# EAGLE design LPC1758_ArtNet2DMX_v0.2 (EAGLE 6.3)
Assembly variants: OHNE USB, OHNE VCC2

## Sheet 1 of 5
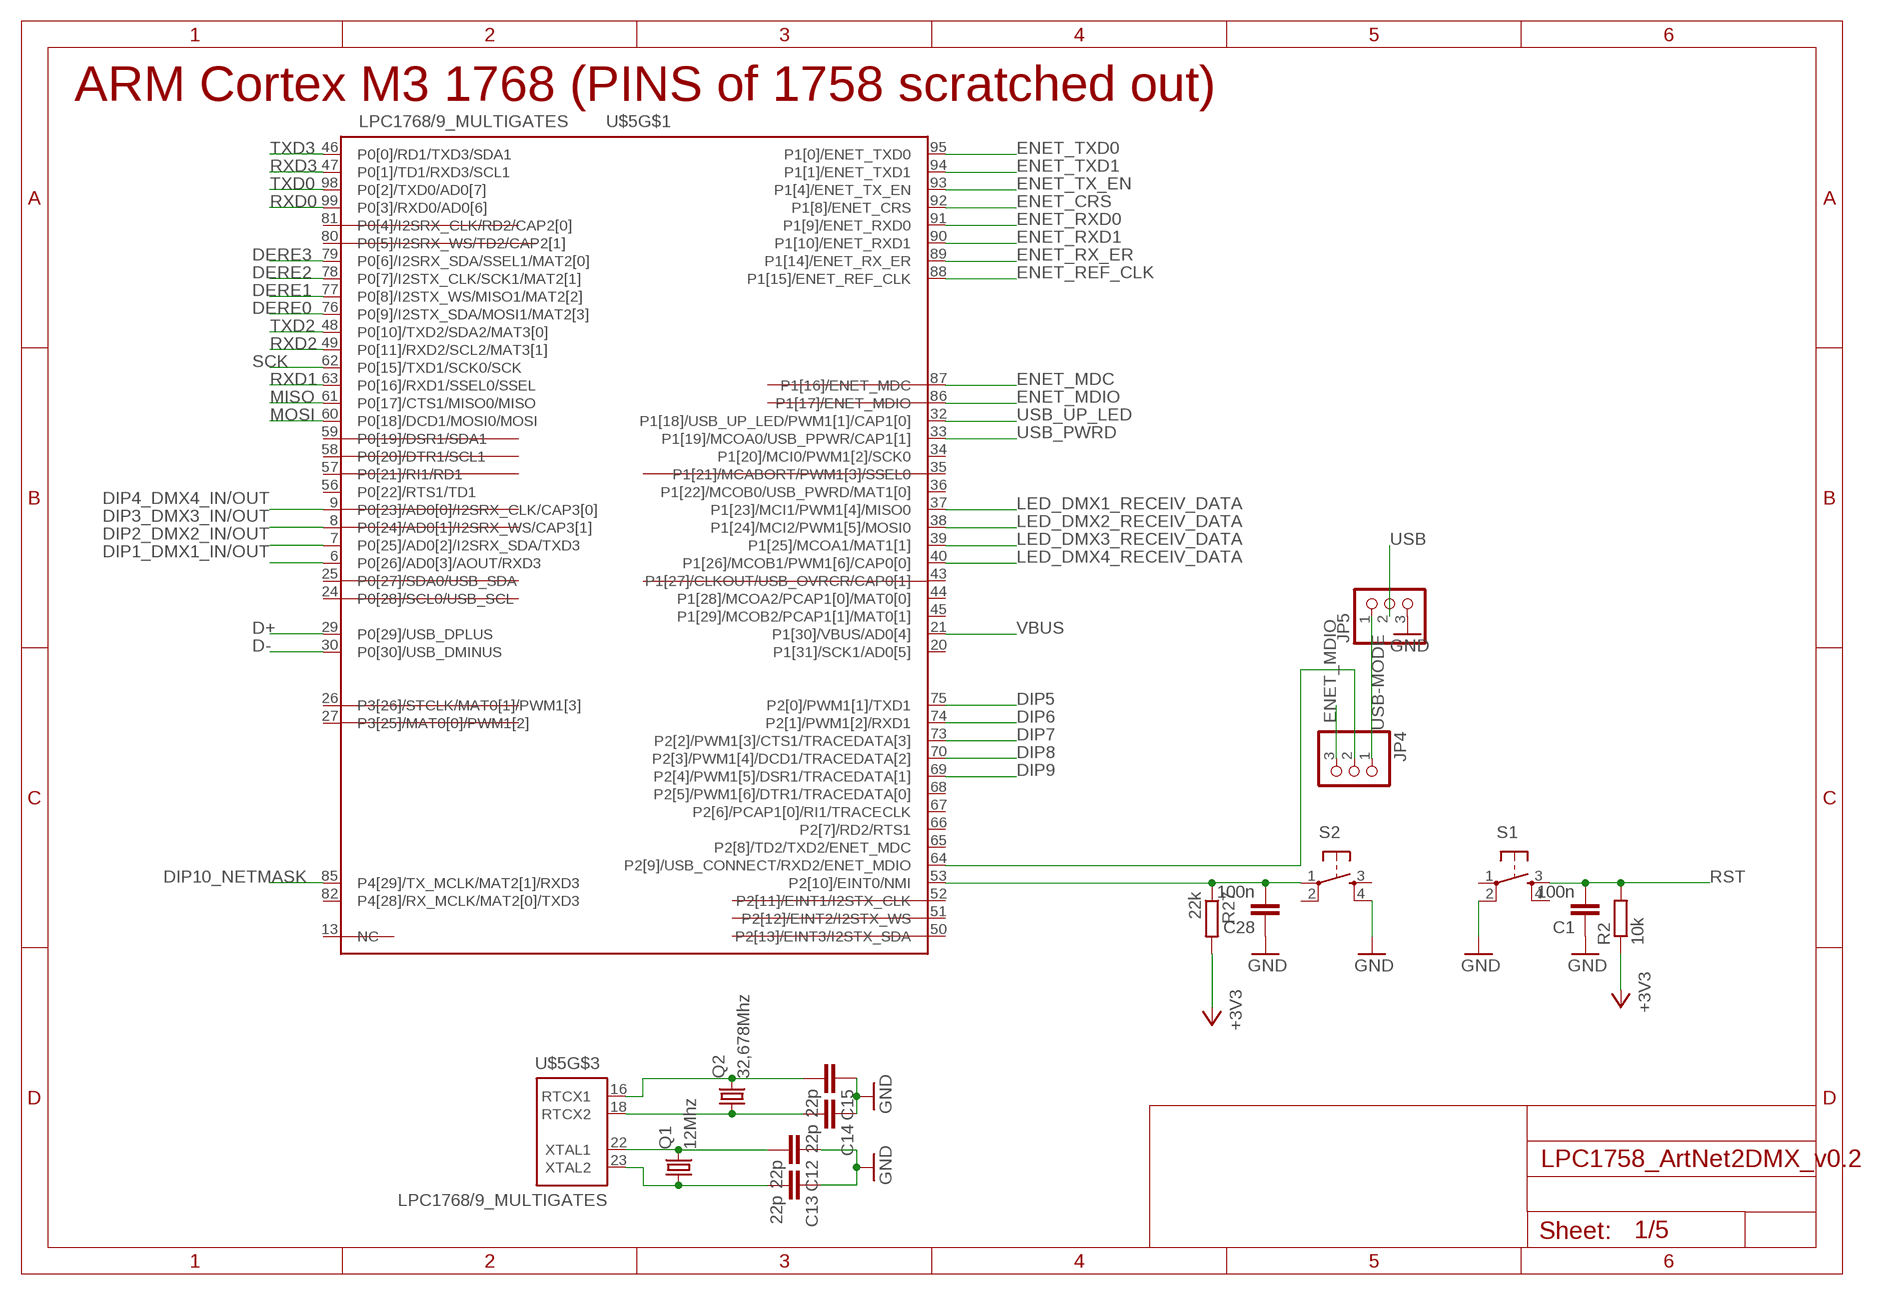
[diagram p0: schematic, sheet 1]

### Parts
C1  100n  C-EUC0805K  [C0805K]
C12  22p  C-EUC0805K  [C0805K]
C13  22p  C-EUC0805K  [C0805K]
C14  22p  C-EUC0805K  [C0805K]
C15  22p  C-EUC0805K  [C0805K]
C28  100n  C-EUC0805K  [C0805K]
JP4  PINHD-1X3_2.54-SMD  [1X03SMD]
JP5  PINHD-1X3_2.54-SMD  [1X03SMD]
Q1  12Mhz  CSM-7X-DU  [CSM-7X-DU]
Q2  32,678Mhz  CSM-7X-DU  [CSM-7X-DU]
R2  10k  R-EU_R0805  [R0805]
R27  22k  R-EU_R0805  [R0805]
S1  TASTER_93XX  [TASTER_93XX]
S2  TASTER_93XX  [TASTER_93XX]
U$5  LPC1768/9_MULTIGATES  [LQFP100-14X14]

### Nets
+3V3: R2.1 R27.2 ; also sheet 2,3,4,5
BUTTON_RESERVE: C28.2 R27.1 S2.1(P) U$5.53(P2[10]/EINT0/NMI)
D+: U$5.29(P0[29]/USB_DPLUS) ; also sheet 4
D-: U$5.30(P0[30]/USB_DMINUS) ; also sheet 4
DERE0: U$5.76(P0[9]/I2STX_SDA/MOSI1/MAT2[3]) ; also sheet 3
DERE1: U$5.77(P0[8]/I2STX_WS/MISO1/MAT2[2]) ; also sheet 3
DERE2: U$5.78(P0[7]/I2STX_CLK/SCK1/MAT2[1]) ; also sheet 3
DERE3: U$5.79(P0[6]/I2SRX_SDA/SSEL1/MAT2[0]) ; also sheet 3
DIP1_DMX1_IN/OUT: U$5.6(P0[26]/AD0[3]/AOUT/RXD3) ; also sheet 3
DIP2_DMX2_IN/OUT: U$5.7(P0[25]/AD0[2]/I2SRX_SDA/TXD3) ; also sheet 3
DIP3_DMX3_IN/OUT: U$5.8(P0[24]/AD0[1]/I2SRX_WS/CAP3[1]) ; also sheet 3
DIP4_DMX4_IN/OUT: U$5.9(P0[23]/AD0[0]/I2SRX_CLK/CAP3[0]) ; also sheet 3
DIP5: U$5.75(P2[0]/PWM1[1]/TXD1) ; also sheet 3
DIP6: U$5.74(P2[1]/PWM1[2]/RXD1) ; also sheet 3
DIP7: U$5.73(P2[2]/PWM1[3]/CTS1/TRACEDATA[3]) ; also sheet 3
DIP8: U$5.70(P2[3]/PWM1[4]/DCD1/TRACEDATA[2]) ; also sheet 3
DIP9: U$5.69(P2[4]/PWM1[5]/DSR1/TRACEDATA[1]) ; also sheet 3
DIP10_NETMASK: U$5.85(P4[29]/TX_MCLK/MAT2[1]/RXD3) ; also sheet 3
ENET_CRS: U$5.92(P1[8]/ENET_CRS) ; also sheet 2
ENET_MDC: U$5.87(P1[16]/ENET_MDC) ; also sheet 2
ENET_MDIO: JP4.3 U$5.86(P1[17]/ENET_MDIO) ; also sheet 2
ENET_MDIO/USB: JP4.2 U$5.64(P2[9]/USB_CONNECT/RXD2/ENET_MDIO)
ENET_REF_CLK: U$5.88(P1[15]/ENET_REF_CLK) ; also sheet 2
ENET_RX_ER: U$5.89(P1[14]/ENET_RX_ER) ; also sheet 2
ENET_RXD0: U$5.91(P1[9]/ENET_RXD0) ; also sheet 2
ENET_RXD1: U$5.90(P1[10]/ENET_RXD1) ; also sheet 2
ENET_TX_EN: U$5.93(P1[4]/ENET_TX_EN) ; also sheet 2
ENET_TXD0: U$5.95(P1[0]/ENET_TXD0) ; also sheet 2
ENET_TXD1: U$5.94(P1[1]/ENET_TXD1) ; also sheet 2
GND: C1.1 C12.1 C13.1 C14.1 C15.1 C28.1 JP5.3 S1.2(P1) S2.4(S1) ; also sheet 2,3,4,5
LED_DMX1_RECEIV_DATA: U$5.37(P1[23]/MCI1/PWM1[4]/MISO0) ; also sheet 3
LED_DMX2_RECEIV_DATA: U$5.38(P1[24]/MCI2/PWM1[5]/MOSI0) ; also sheet 3
LED_DMX3_RECEIV_DATA: U$5.39(P1[25]/MCOA1/MAT1[1]) ; also sheet 3
LED_DMX4_RECEIV_DATA: U$5.40(P1[26]/MCOB1/PWM1[6]/CAP0[0]) ; also sheet 3
MISO: U$5.61(P0[17]/CTS1/MISO0/MISO) ; also sheet 5
MOSI: U$5.60(P0[18]/DCD1/MOSI0/MOSI) ; also sheet 5
N$12: C12.2 Q1.2 U$5.22(XTAL1)
N$13: C13.2 Q1.1 U$5.23(XTAL2)
N$16: C14.2 Q2.1 U$5.18(RTCX2)
N$20: C15.2 Q2.2 U$5.16(RTCX1)
RST: C1.2 R2.2 S1.3(S) ; also sheet 2,5
RXD0: U$5.99(P0[3]/RXD0/AD0[6]) ; also sheet 3
RXD1: U$5.63(P0[16]/RXD1/SSEL0/SSEL) ; also sheet 3
RXD2: U$5.49(P0[11]/RXD2/SCL2/MAT3[1]) ; also sheet 3
RXD3: U$5.47(P0[1]/TD1/RXD3/SCL1) ; also sheet 3
SCK: U$5.62(P0[15]/TXD1/SCK0/SCK) ; also sheet 5
TXD0: U$5.98(P0[2]/TXD0/AD0[7]) ; also sheet 3
TXD2: U$5.48(P0[10]/TXD2/SDA2/MAT3[0]) ; also sheet 3
TXD3: U$5.46(P0[0]/RD1/TXD3/SDA1) ; also sheet 3
USB: JP5.2 ; also sheet 4
USB-MODE: JP4.1 JP5.1
USB_PWRD: U$5.33(P1[19]/MCOA0/USB_PPWR/CAP1[1]) ; also sheet 4
USB_UP_LED: U$5.32(P1[18]/USB_UP_LED/PWM1[1]/CAP1[0]) ; also sheet 4
VBUS: U$5.21(P1[30]/VBUS/AD0[4]) ; also sheet 4
Unconnected: S1.1(P) S1.4(S1) S2.2(P1) S2.3(S) U$5.13(NC) U$5.20(P1[31]/SCK1/AD0[5]) U$5.24(P0[28]/SCL0/USB_SCL) U$5.25(P0[27]/SDA0/USB_SDA) U$5.26(P3[26]/STCLK/MAT0[1]/PWM1[3]) U$5.27(P3[25]/MAT0[0]/PWM1[2]) U$5.34(P1[20]/MCI0/PWM1[2]/SCK0) U$5.35(P1[21]/MCABORT/PWM1[3]/SSEL0) U$5.36(P1[22]/MCOB0/USB_PWRD/MAT1[0]) U$5.43(P1[27]/CLKOUT/USB_OVRCR/CAP0[1]) U$5.44(P1[28]/MCOA2/PCAP1[0]/MAT0[0]) U$5.45(P1[29]/MCOB2/PCAP1[1]/MAT0[1]) U$5.50(P2[13]/EINT3/I2STX_SDA) U$5.51(P2[12]/EINT2/I2STX_WS) U$5.52(P2[11]/EINT1/I2STX_CLK) U$5.56(P0[22]/RTS1/TD1) U$5.57(P0[21]/RI1/RD1) U$5.58(P0[20]/DTR1/SCL1) U$5.59(P0[19]/DSR1/SDA1) U$5.65(P2[8]/TD2/TXD2/ENET_MDC) U$5.66(P2[7]/RD2/RTS1) U$5.67(P2[6]/PCAP1[0]/RI1/TRACECLK) U$5.68(P2[5]/PWM1[6]/DTR1/TRACEDATA[0]) U$5.80(P0[5]/I2SRX_WS/TD2/CAP2[1]) U$5.81(P0[4]/I2SRX_CLK/RD2/CAP2[0]) U$5.82(P4[28]/RX_MCLK/MAT2[0]/TXD3)

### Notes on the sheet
- ARM Cortex M3 1768 (PINS of 1758 scratched out)

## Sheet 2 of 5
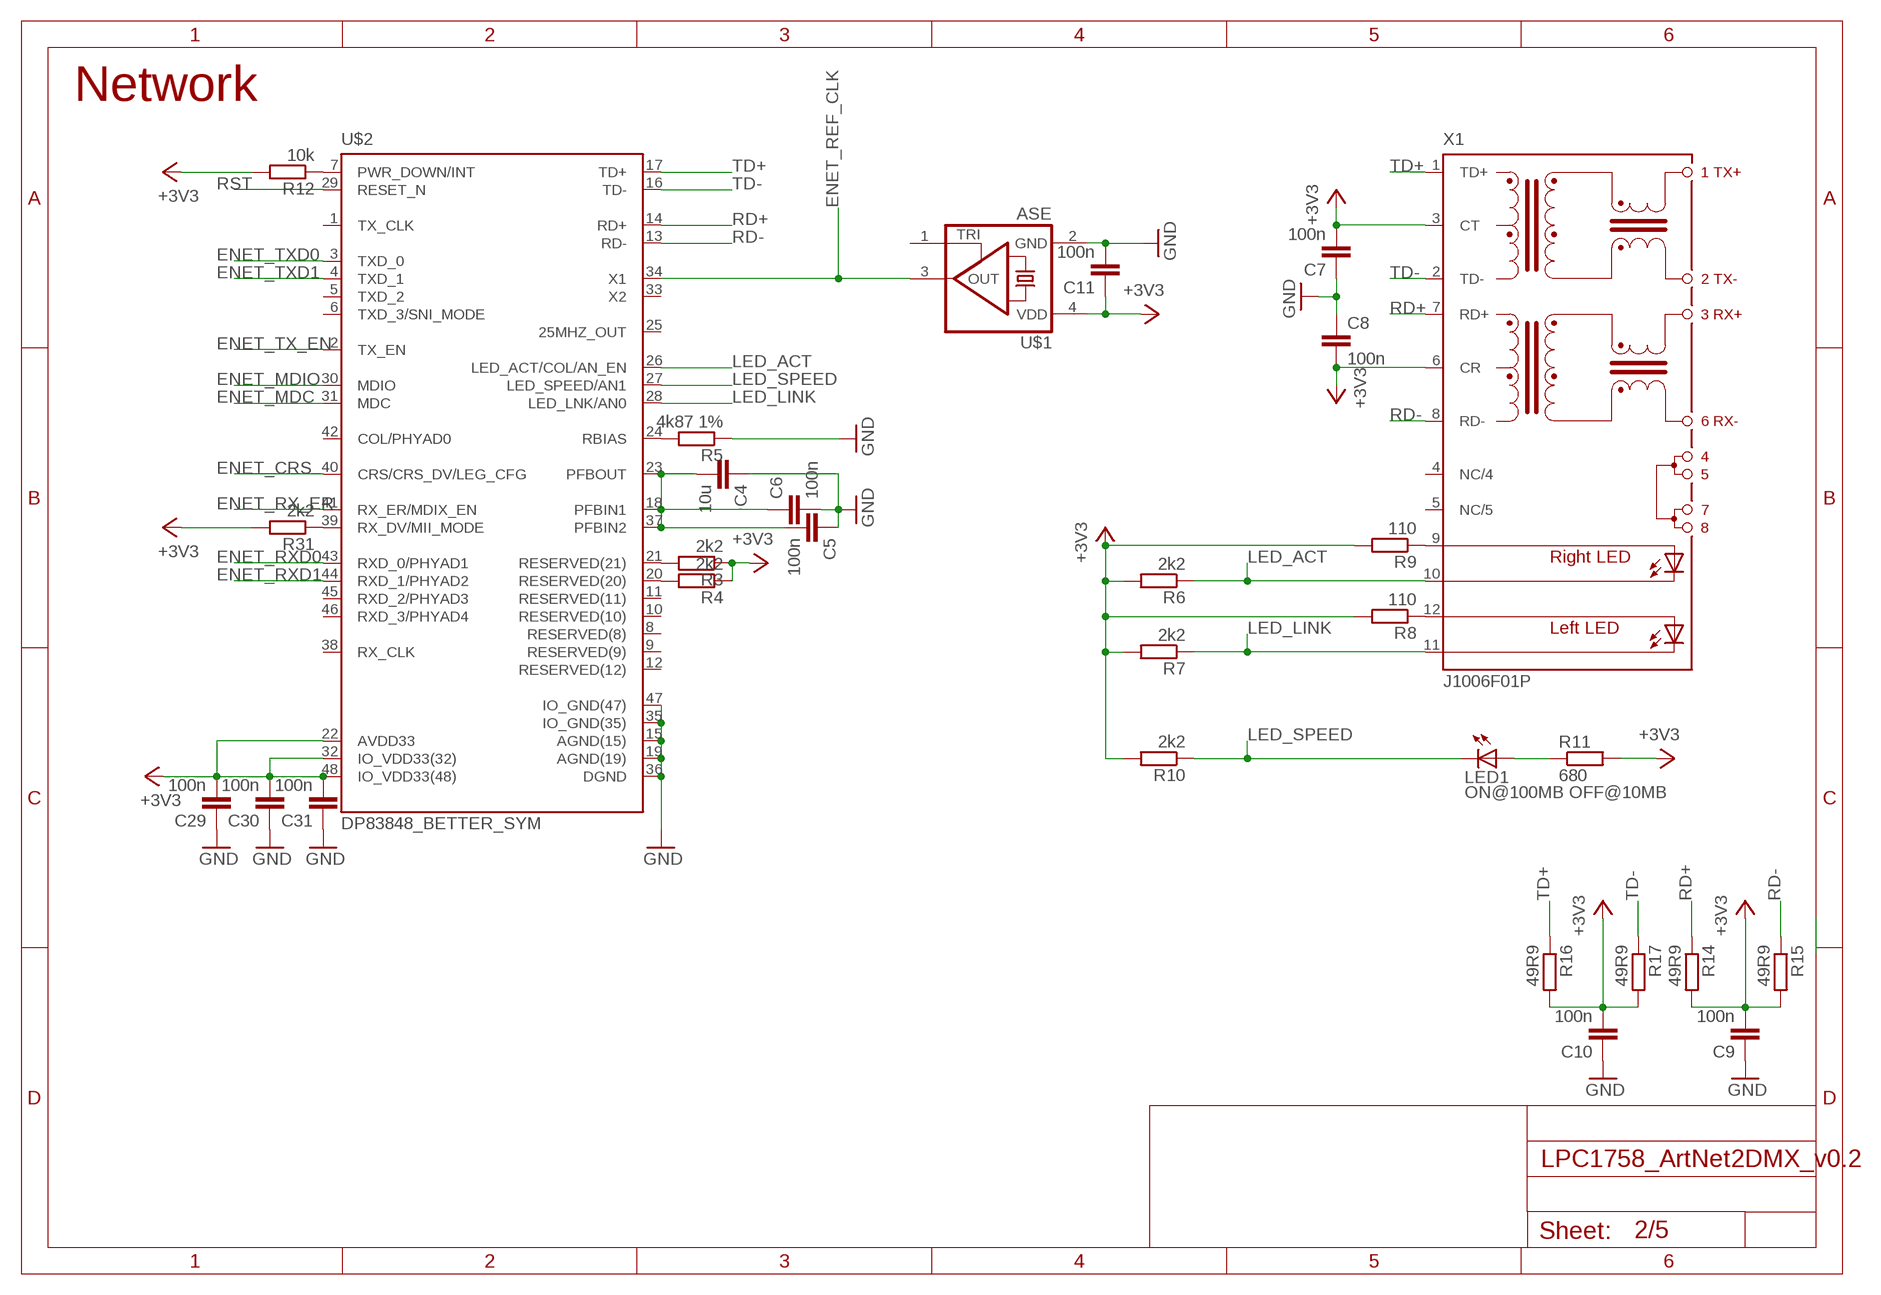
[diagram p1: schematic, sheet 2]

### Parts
C4  10u  C-EUC0805K  [C0805K]
C5  100n  C-EUC0805K  [C0805K]
C6  100n  C-EUC0805K  [C0805K]
C7  100n  C-EUC0805K  [C0805K]
C8  100n  C-EUC0805K  [C0805K]
C9  100n  C-EUC0805K  [C0805K]
C10  100n  C-EUC0805K  [C0805K]
C11  100n  C-EUC0805K  [C0805K]
C29  100n  C-EUC0805K  [C0805K]
C30  100n  C-EUC0805K  [C0805K]
C31  100n  C-EUC0805K  [C0805K]
LED1  ON@100MB OFF@10MB  LEDCHIP-LED0805  [CHIP-LED0805]
R3  2k2  R-EU_R0805  [R0805]
R4  2k2  R-EU_R0805  [R0805]
R5  4k87 1%  R-EU_R0805  [R0805]
R6  2k2  R-EU_R0805  [R0805]
R7  2k2  R-EU_R0805  [R0805]
R8  110  R-EU_R0805  [R0805]
R9  110  R-EU_R0805  [R0805]
R10  2k2  R-EU_R0805  [R0805]
R11  680  R-EU_R0805  [R0805]
R12  10k  R-EU_R0805  [R0805]
R14  49R9  R-EU_R0805  [R0805]
R15  49R9  R-EU_R0805  [R0805]
R16  49R9  R-EU_R0805  [R0805]
R17  49R9  R-EU_R0805  [R0805]
R31  2k2  R-EU_R0805  [R0805]
U$1  ASE  [ASE]
U$2  DP83848_BETTER_SYM  [LQFP48]
X1  J1006F01P  [J1]

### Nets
+3V3: C7.2 C8.2 C9.2 C10.2 C11.1 C29.2 C30.2 C31.2 R3.1 R4.1 R6.2 R7.2 R8.2 R9.2 R10.2 R11.2 R12.2 R14.2 R15.2 R16.2 R17.2 R31.2 U$1.4(VDD) U$2.22(AVDD33) U$2.32(IO_VDD33(32)) U$2.48(IO_VDD33(48)) X1.3(CT) X1.6(CR) ; also sheet 1,3,4,5
ENET_CRS: U$2.40(CRS/CRS_DV/LEG_CFG) ; also sheet 1
ENET_MDC: U$2.31(MDC) ; also sheet 1
ENET_MDIO: U$2.30(MDIO) ; also sheet 1
ENET_REF_CLK: U$1.3(OUT) U$2.34(X1) ; also sheet 1
ENET_RX_ER: U$2.41(RX_ER/MDIX_EN) ; also sheet 1
ENET_RXD0: U$2.43(RXD_0/PHYAD1) ; also sheet 1
ENET_RXD1: U$2.44(RXD_1/PHYAD2) ; also sheet 1
ENET_TX_EN: U$2.2(TX_EN) ; also sheet 1
ENET_TXD0: U$2.3(TXD_0) ; also sheet 1
ENET_TXD1: U$2.4(TXD_1) ; also sheet 1
GND: C4.1 C5.1 C6.2 C7.1 C8.1 C9.1 C10.1 C11.2 C29.1 C30.1 C31.1 R5.1 U$1.2(GND) U$2.15(AGND(15)) U$2.19(AGND(19)) U$2.35(IO_GND(35)) U$2.36(DGND) U$2.47(IO_GND(47)) ; also sheet 1,3,4,5
LED_ACT: R6.1 U$2.26(LED_ACT/COL/AN_EN) X1.10(C-R)
LED_LINK: R7.1 U$2.28(LED_LNK/AN0) X1.11(C-L)
LED_SPEED: LED1.C R10.1 U$2.27(LED_SPEED/AN1)
N$4: R8.1 X1.12(A-L)
N$8: R9.1 X1.9(A-R)
N$9: LED1.A R11.1
N$10: R12.1 U$2.7(PWR_DOWN/INT)
N$14: R3.2 U$2.21(RESERVED(21))
N$15: R4.2 U$2.20(RESERVED(20))
N$17: C4.2 C5.2 C6.1 U$2.18(PFBIN1) U$2.23(PFBOUT) U$2.37(PFBIN2)
N$18: R5.2 U$2.24(RBIAS)
N$19: R31.1 U$2.39(RX_DV/MII_MODE)
RD+: R14.1 U$2.14(RD+) X1.7(RD+)
RD-: R15.1 U$2.13(RD-) X1.8(RD-)
RST: U$2.29(RESET_N) ; also sheet 1,5
TD+: R16.1 U$2.17(TD+) X1.1(TD+)
TD-: R17.1 U$2.16(TD-) X1.2(TD-)
Unconnected: U$1.1(TRI) U$2.1(TX_CLK) U$2.5(TXD_2) U$2.6(TXD_3/SNI_MODE) U$2.8(RESERVED(8)) U$2.9(RESERVED(9)) U$2.10(RESERVED(10)) U$2.11(RESERVED(11)) U$2.12(RESERVED(12)) U$2.25(25MHZ_OUT) U$2.33(X2) U$2.38(RX_CLK) U$2.42(COL/PHYAD0) U$2.45(RXD_2/PHYAD3) U$2.46(RXD_3/PHYAD4) X1.4(NC/4) X1.5(NC/5)

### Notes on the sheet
- Network

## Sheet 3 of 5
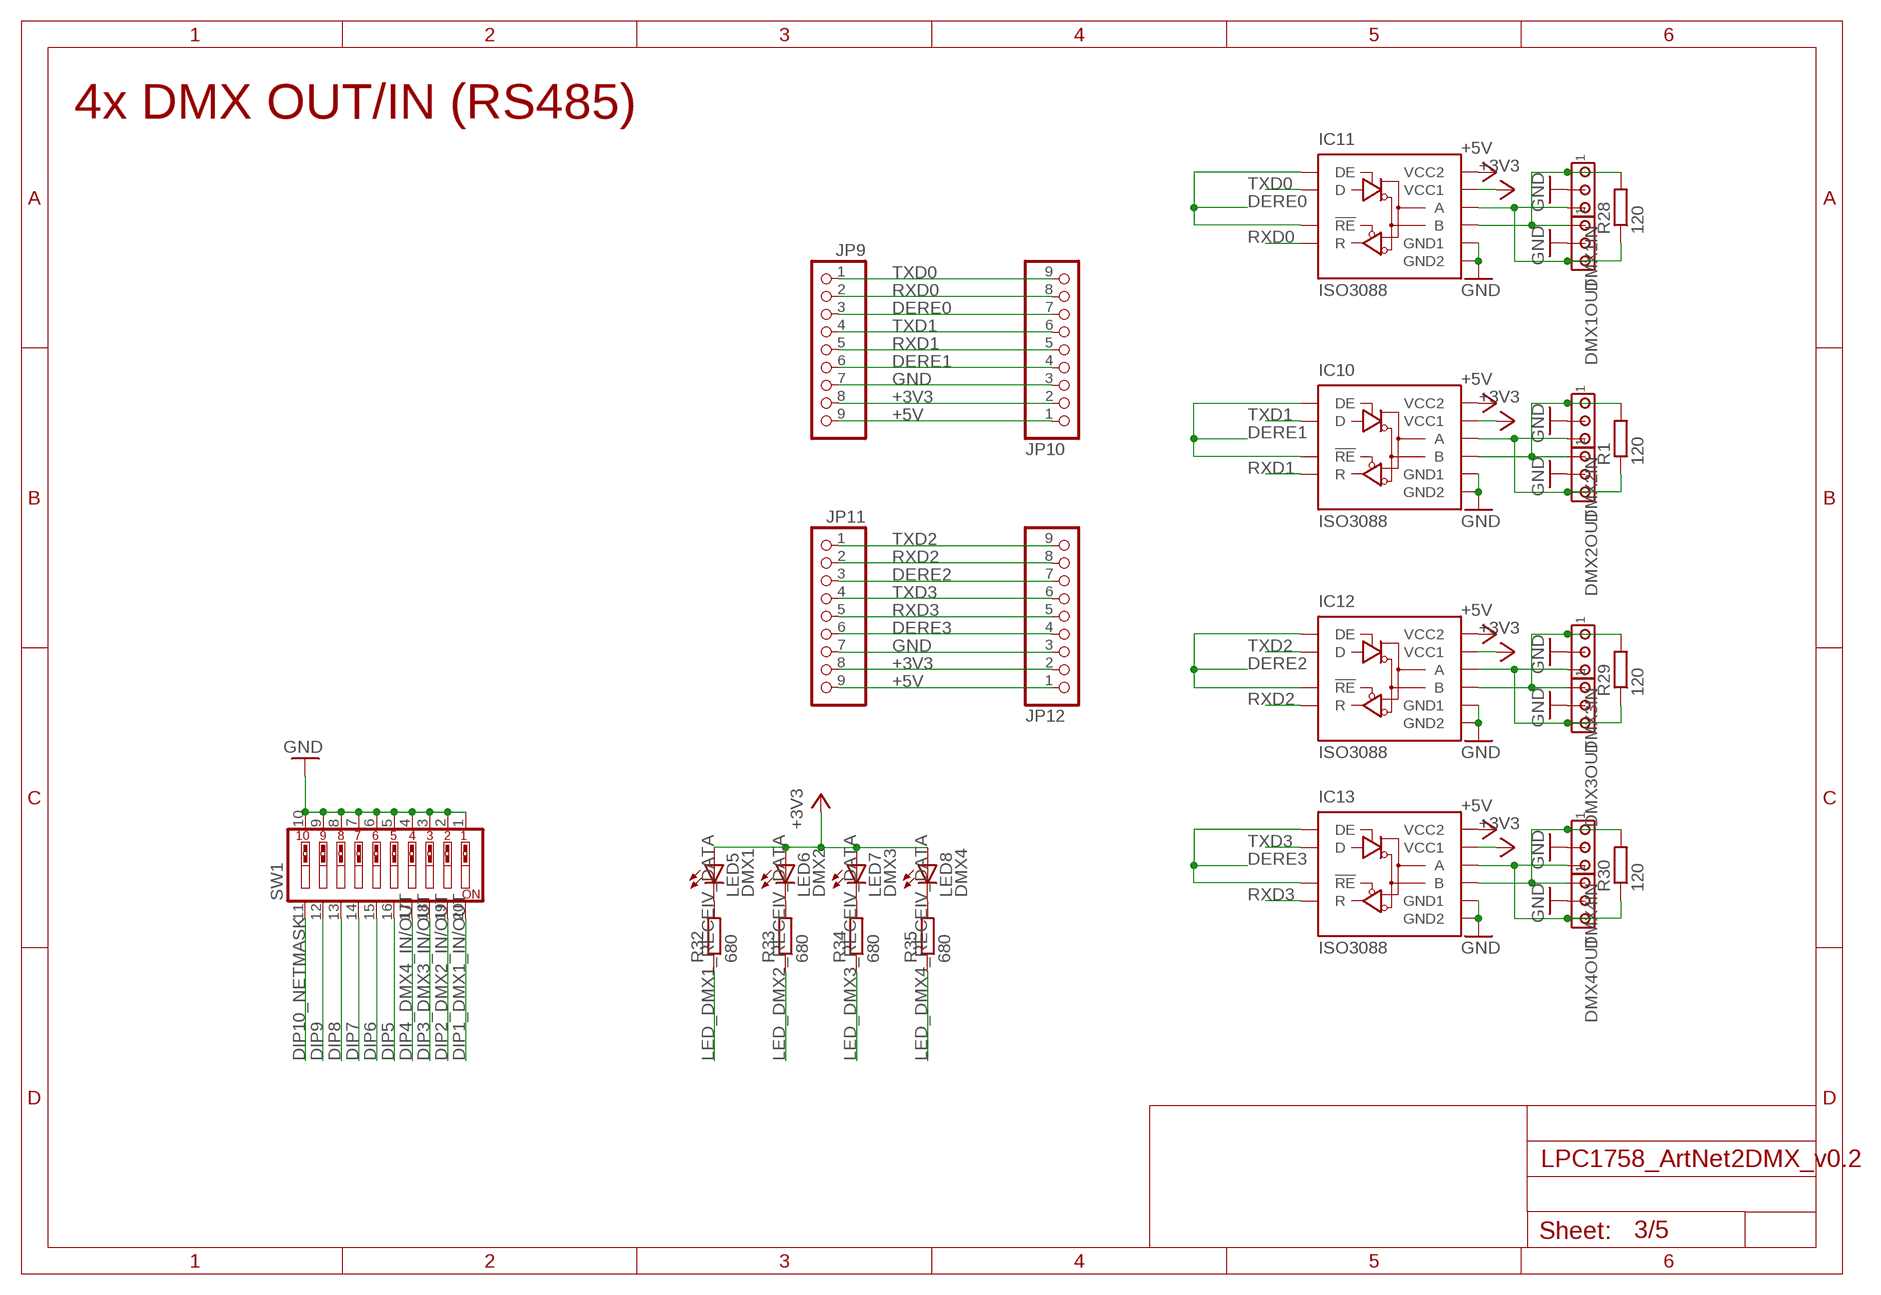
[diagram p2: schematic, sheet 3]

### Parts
DMX1IN  MTA03-100  [10X03MTA]
DMX1OUT  MTA03-100  [10X03MTA]
DMX2IN  MTA03-100  [10X03MTA]
DMX2OUT  MTA03-100  [10X03MTA]
DMX3IN  MTA03-100  [10X03MTA]
DMX3OUT  MTA03-100  [10X03MTA]
DMX4IN  MTA03-100  [10X03MTA]
DMX4OUT  MTA03-100  [10X03MTA]
IC10  ISO3088  [SO16]
IC11  ISO3088  [SO16]
IC12  ISO3088  [SO16]
IC13  ISO3088  [SO16]
JP9  PINHD-1X9_2.54  [1X09]
JP10  PINHD-1X9_2.54-SMD  [1X09SMD]
JP11  PINHD-1X9_2.54  [1X09]
JP12  PINHD-1X9_2.54-SMD  [1X09SMD]
LED5  DMX1  LEDCHIP-LED0805  [CHIP-LED0805]
LED6  DMX2  LEDCHIP-LED0805  [CHIP-LED0805]
LED7  DMX3  LEDCHIP-LED0805  [CHIP-LED0805]
LED8  DMX4  LEDCHIP-LED0805  [CHIP-LED0805]
R1  120  R-EU_R0805  [R0805]
R28  120  R-EU_R0805  [R0805]
R29  120  R-EU_R0805  [R0805]
R30  120  R-EU_R0805  [R0805]
R32  680  R-EU_R0805  [R0805]
R33  680  R-EU_R0805  [R0805]
R34  680  R-EU_R0805  [R0805]
R35  680  R-EU_R0805  [R0805]
SW1  SW_DIP-10  [EDG-10]

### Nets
+3V3: IC10.1(VCC1) IC11.1(VCC1) IC12.1(VCC1) IC13.1(VCC1) JP9.8 JP10.2 JP11.8 JP12.2 LED5.A LED6.A LED7.A LED8.A ; also sheet 1,2,4,5
+5V: IC10.16(VCC2) IC11.16(VCC2) IC12.16(VCC2) IC13.16(VCC2) JP9.9 JP10.1 JP11.9 JP12.1 ; also sheet 4,5
DERE0: IC11.4(!RE) IC11.5(DE) JP9.3 JP10.7 ; also sheet 1
DERE1: IC10.4(!RE) IC10.5(DE) JP9.6 JP10.4 ; also sheet 1
DERE2: IC12.4(!RE) IC12.5(DE) JP11.3 JP12.7 ; also sheet 1
DERE3: IC13.4(!RE) IC13.5(DE) JP11.6 JP12.4 ; also sheet 1
DIP1_DMX1_IN/OUT: SW1.20 ; also sheet 1
DIP2_DMX2_IN/OUT: SW1.19 ; also sheet 1
DIP3_DMX3_IN/OUT: SW1.18 ; also sheet 1
DIP4_DMX4_IN/OUT: SW1.17 ; also sheet 1
DIP5: SW1.16 ; also sheet 1
DIP6: SW1.15 ; also sheet 1
DIP7: SW1.14 ; also sheet 1
DIP8: SW1.13 ; also sheet 1
DIP9: SW1.12 ; also sheet 1
DIP10_NETMASK: SW1.11 ; also sheet 1
GND: DMX1IN.2 DMX1OUT.2 DMX2IN.2 DMX2OUT.2 DMX3IN.2 DMX3OUT.2 DMX4IN.2 DMX4OUT.2 IC10.2(GND1) IC10.7(GND1) IC10.8(GND1) IC10.9(GND2) IC10.10(GND2) IC10.15(GND2) IC11.2(GND1) IC11.7(GND1) IC11.8(GND1) IC11.9(GND2) IC11.10(GND2) IC11.15(GND2) IC12.2(GND1) IC12.7(GND1) IC12.8(GND1) IC12.9(GND2) IC12.10(GND2) IC12.15(GND2) IC13.2(GND1) IC13.7(GND1) IC13.8(GND1) IC13.9(GND2) IC13.10(GND2) IC13.15(GND2) JP9.7 JP10.3 JP11.7 JP12.3 SW1.1 SW1.2 SW1.3 SW1.4 SW1.5 SW1.6 SW1.7 SW1.8 SW1.9 SW1.10 ; also sheet 1,2,4,5
LED_DMX1_RECEIV_DATA: R32.1 ; also sheet 1
LED_DMX2_RECEIV_DATA: R33.1 ; also sheet 1
LED_DMX3_RECEIV_DATA: R34.1 ; also sheet 1
LED_DMX4_RECEIV_DATA: R35.1 ; also sheet 1
N$1: DMX2IN.3 DMX2OUT.3 IC10.12(A) R1.1
N$2: DMX2IN.1 DMX2OUT.1 IC10.13(B) R1.2
N$5: LED5.C R32.2
N$6: LED6.C R33.2
N$36: DMX1IN.3 DMX1OUT.3 IC11.12(A) R28.1
N$37: DMX1IN.1 DMX1OUT.1 IC11.13(B) R28.2
N$38: DMX3IN.3 DMX3OUT.3 IC12.12(A) R29.1
N$39: DMX3IN.1 DMX3OUT.1 IC12.13(B) R29.2
N$40: DMX4IN.3 DMX4OUT.3 IC13.12(A) R30.1
N$41: DMX4IN.1 DMX4OUT.1 IC13.13(B) R30.2
N$44: LED7.C R34.2
N$45: LED8.C R35.2
RXD0: IC11.3(R) JP9.2 JP10.8 ; also sheet 1
RXD1: IC10.3(R) JP9.5 JP10.5 ; also sheet 1
RXD2: IC12.3(R) JP11.2 JP12.8 ; also sheet 1
RXD3: IC13.3(R) JP11.5 JP12.5 ; also sheet 1
TXD0: IC11.6(D) JP9.1 JP10.9 ; also sheet 1
TXD1: IC10.6(D) JP9.4 JP10.6
TXD2: IC12.6(D) JP11.1 JP12.9 ; also sheet 1
TXD3: IC13.6(D) JP11.4 JP12.6 ; also sheet 1

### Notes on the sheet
- 4x DMX OUT/IN (RS485)

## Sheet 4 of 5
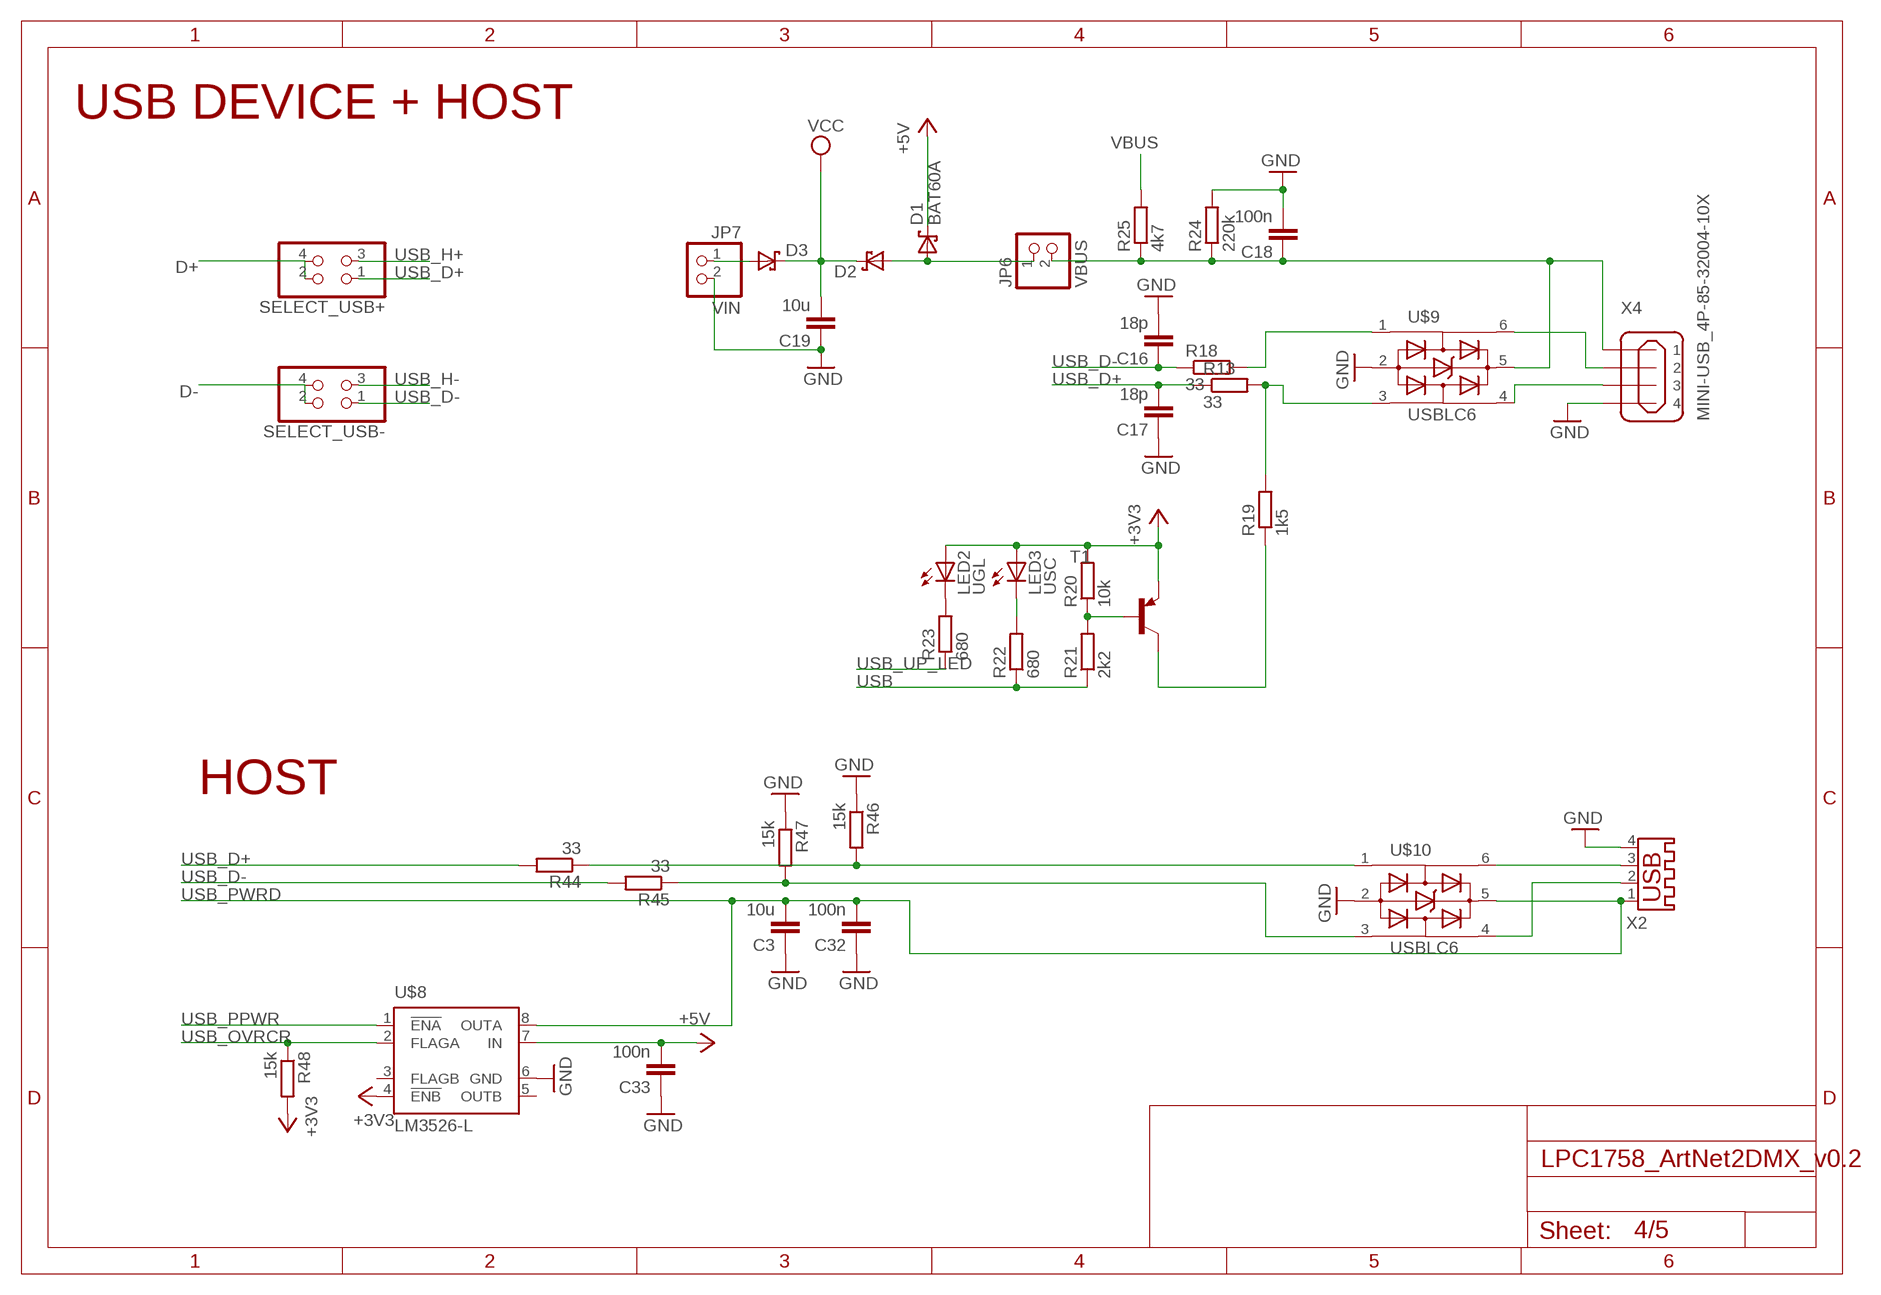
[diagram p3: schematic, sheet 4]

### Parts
C3  10u  C-EUC0805K  [C0805K]  (not fitted in variant OHNE USB)
C16  18p  C-EUC0805K  [C0805K]  (not fitted in variant OHNE USB)
C17  18p  C-EUC0805K  [C0805K]  (not fitted in variant OHNE USB)
C18  100n  C-EUC0805K  [C0805K]  (not fitted in variant OHNE USB)
C19  10u  C-EUC0805K  [C0805K]  (not fitted in variant OHNE USB)
C32  100n  C-EUC0805K  [C0805K]  (not fitted in variant OHNE USB)
C33  100n  C-EUC0805K  [C0805K]  (not fitted in variant OHNE USB)
D1  BAT60A  [BAT60A]  (not fitted in variant OHNE USB)
D2  BAT60A  [BAT60A]  (not fitted in variant OHNE USB)
D3  BAT60A  [BAT60A]  (not fitted in variant OHNE USB)
JP6  VBUS  PINHD-1X2_2.54-SMD  [1X02SMD]  (not fitted in variant OHNE USB)
JP7  VIN  PINHD-1X2_2.54-SMD  [1X02SMD]  (not fitted in variant OHNE USB)
LED2  UGL  LEDCHIP-LED0805  [CHIP-LED0805]  (not fitted in variant OHNE USB)
LED3  USC  LEDCHIP-LED0805  [CHIP-LED0805]  (not fitted in variant OHNE USB)
R13  33  R-EU_R0805  [R0805]  (not fitted in variant OHNE USB)
R18  33  R-EU_R0805  [R0805]  (not fitted in variant OHNE USB)
R19  1k5  R-EU_R0805  [R0805]  (not fitted in variant OHNE USB)
R20  10k  R-EU_R0805  [R0805]  (not fitted in variant OHNE USB)
R21  2k2  R-EU_R0805  [R0805]  (not fitted in variant OHNE USB)
R22  680  R-EU_R0805  [R0805]  (not fitted in variant OHNE USB)
R23  680  R-EU_R0805  [R0805]  (not fitted in variant OHNE USB)
R24  220k  R-EU_R0805  [R0805]  (not fitted in variant OHNE USB)
R25  4k7  R-EU_R0805  [R0805]  (not fitted in variant OHNE USB)
R44  33  R-EU_R0805  [R0805]  (not fitted in variant OHNE USB)
R45  33  R-EU_R0805  [R0805]  (not fitted in variant OHNE USB)
R46  15k  R-EU_R0805  [R0805]  (not fitted in variant OHNE USB)
R47  15k  R-EU_R0805  [R0805]  (not fitted in variant OHNE USB)
R48  15k  R-EU_R0805  [R0805]  (not fitted in variant OHNE USB)
SELECT_USB+  PINHD-2X2_2.54-SMD  [2X02SMD]  (not fitted in variant OHNE USB)
SELECT_USB-  PINHD-2X2_2.54-SMD  [2X02SMD]  (not fitted in variant OHNE USB)
T1  BC857B-PNP-SOT23-BEC  [SOT23-BEC]  (not fitted in variant OHNE USB)
U$8  LM3526-L  [SO08]  (not fitted in variant OHNE USB)
U$9  USBLC6  [SOT23-6]  (not fitted in variant OHNE USB)
U$10  USBLC6  [SOT23-6]  (not fitted in variant OHNE USB)
X2  USB-A003  [USB-A003]  (not fitted in variant OHNE USB)
X4  MINI-USB_4P-85-32004-10X  [85-32004-10X]  (not fitted in variant OHNE USB)

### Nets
+3V3: LED2.A LED3.A R20.2 R48.2 T1.E U$8.4(!ENB) ; also sheet 1,2,3,5
+5V: C33.2 D1.P$1(K) U$8.7(IN) ; also sheet 3,5
D+: SELECT_USB+.2 SELECT_USB+.4 ; also sheet 1
D-: SELECT_USB-.2 SELECT_USB-.4 ; also sheet 1
GND: C3.1 C16.2 C17.1 C18.2 C19.1 C32.1 C33.1 JP7.2 R24.2 R46.1 R47.1 U$8.6(GND) U$9.2(GND) U$10.2(GND) X2.4 X4.4 ; also sheet 1,2,3,5
N$21: U$9.6(I/O1_2) X4.2
N$22: U$9.4(I/O2_2) X4.3
N$23: R45.1 R47.2 U$10.3(I/O2_1)
N$24: R13.2 R19.2 U$9.3(I/O2_1)
N$25: R44.1 R46.2 U$10.1(I/O1_1)
N$26: R19.1 T1.C
N$27: LED2.C R23.2
N$28: R20.1 R21.2 T1.B
N$29: LED3.C R22.2
N$30: C18.1 JP6.2 R24.1 R25.1 U$9.5(VBUS) X4.1
N$31: D1.P$2(A) D2.P$2(A) JP6.1
N$33: D3.P$2(A) JP7.1
N$34: R18.2 U$9.1(I/O1_1)
N$47: U$10.4(I/O2_2) X2.2
N$48: U$10.6(I/O1_2) X2.3
USB: R21.1 R22.1 ; also sheet 1
USB_D+: C17.2 R13.1 R44.2 SELECT_USB+.1
USB_D-: C16.1 R18.1 R45.2 SELECT_USB-.1
USB_H+: SELECT_USB+.3
USB_H-: SELECT_USB-.3
USB_OVRCR: R48.1 U$8.2(FLAGA)
USB_PPWR: U$8.1(!ENA)
USB_PWRD: C3.2 C32.2 U$8.8(OUTA) U$10.5(VBUS) X2.1 ; also sheet 1
USB_UP_LED: R23.1 ; also sheet 1
VBUS: R25.2 ; also sheet 1
VCC: C19.2 D2.P$1(K) D3.P$1(K) ; also sheet 5
Unconnected: U$8.3(FLAGB) U$8.5(OUTB)

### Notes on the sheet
- USB DEVICE + HOST
- HOST

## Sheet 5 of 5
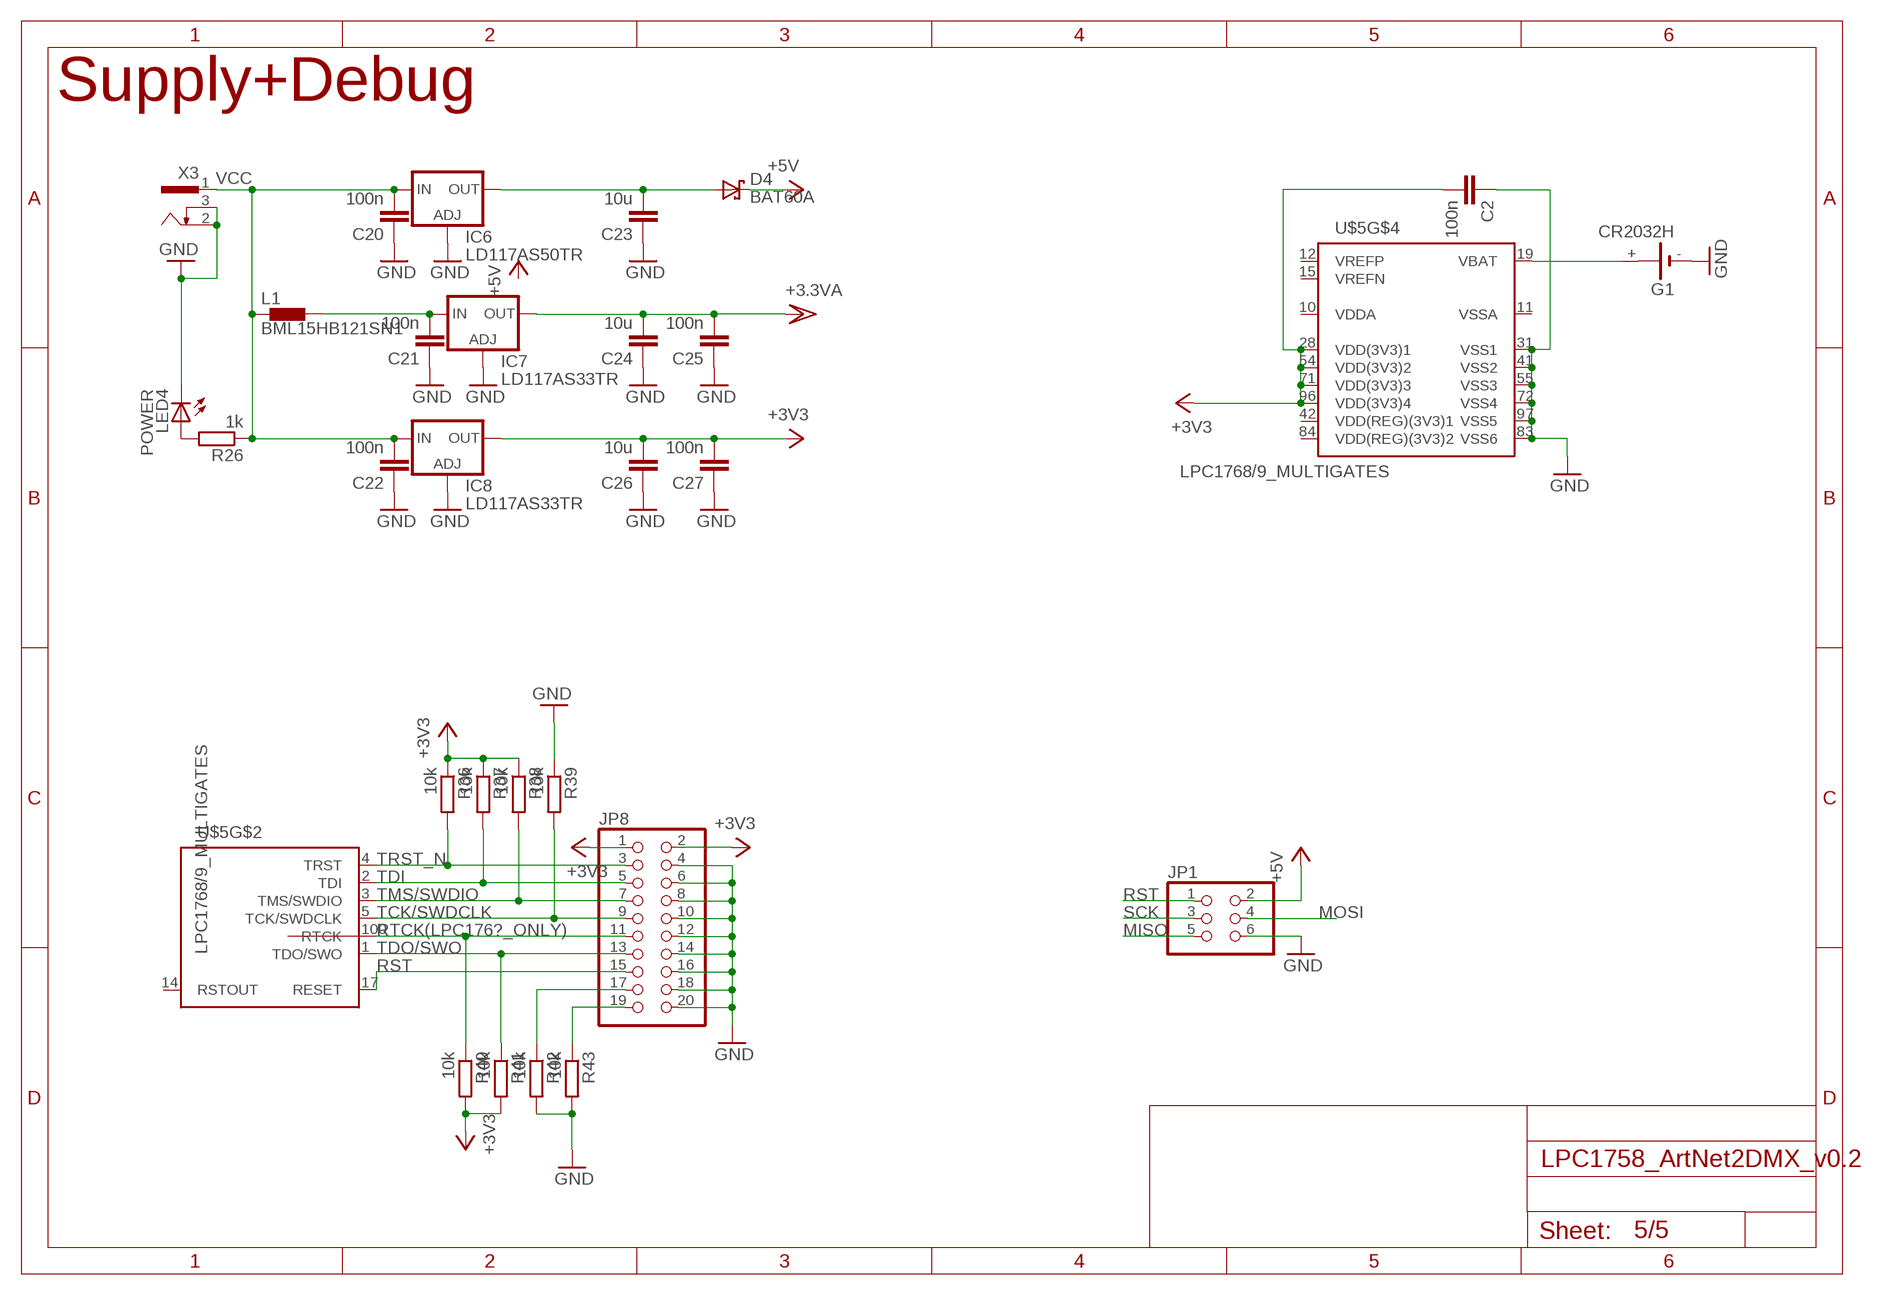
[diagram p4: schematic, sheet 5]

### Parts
C2  100n  C-EUC0805K  [C0805K]
C20  100n  C-EUC0805K  [C0805K]
C21  100n  C-EUC0805K  [C0805K]  (not fitted in variant OHNE VCC2)
C22  100n  C-EUC0805K  [C0805K]
C23  10u  C-EUC0805K  [C0805K]
C24  10u  C-EUC0805K  [C0805K]  (not fitted in variant OHNE VCC2)
C25  100n  C-EUC0805K  [C0805K]  (not fitted in variant OHNE VCC2)
C26  10u  C-EUC0805K  [C0805K]
C27  100n  C-EUC0805K  [C0805K]
D4  BAT60A  [BAT60A]
G1  CR2032H  [CR2032H]
IC6  LD117AS50TR  [SOT223]
IC7  LD117AS33TR  [SOT223]  (not fitted in variant OHNE VCC2)
IC8  LD117AS33TR  [SOT223]
JP1  PINHD-2X3_2.54-SMD  [2X03SMD]
JP8  PINHD-2X10_2,54-90°_SEMI_SMD  [2X10SMD-90_2SIDES]
L1  BML15HB121SN1  [0402]  (not fitted in variant OHNE VCC2)
LED4  POWER  LEDCHIP-LED0805  [CHIP-LED0805]
R26  1k  R-EU_R0805  [R0805]
R36  10k  R-EU_R0805  [R0805]
R37  10k  R-EU_R0805  [R0805]
R38  10k  R-EU_R0805  [R0805]
R39  10k  R-EU_R0805  [R0805]
R40  10k  R-EU_R0805  [R0805]
R41  10k  R-EU_R0805  [R0805]
R42  10k  R-EU_R0805  [R0805]
R43  10k  R-EU_R0805  [R0805]
X3  733980-62  [733980-62]

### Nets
+3.3VA: C24.2 C25.2 IC7.4(OUT)
+3V3: C2.2 C26.2 C27.2 IC8.4(OUT) JP8.1 JP8.2 R36.1 R37.1 R38.1 R40.2 R41.2 U$5.28(VDD(3V3)1) U$5.54(VDD(3V3)2) U$5.71(VDD(3V3)3) U$5.96(VDD(3V3)4) ; also sheet 1,2,3,4
+5V: D4.P$1(K) JP1.2 ; also sheet 3,4
GND: C2.1 C20.1 C21.1 C22.1 C23.1 C24.1 C25.1 C26.1 C27.1 G1.- IC6.1(ADJ) IC7.1(ADJ) IC8.1(ADJ) JP1.6 JP8.4 JP8.6 JP8.8 JP8.10 JP8.12 JP8.14 JP8.16 JP8.18 JP8.20 LED4.C R39.1 R42.2 R43.2 U$5.31(VSS1) U$5.41(VSS2) U$5.55(VSS3) U$5.72(VSS4) U$5.83(VSS6) U$5.97(VSS5) X3.2 X3.3 ; also sheet 1,2,3,4
MISO: JP1.5 ; also sheet 1
MOSI: JP1.4 ; also sheet 1
N$11: C21.2 IC7.3(IN) L1.2
N$32: LED4.A R26.2
N$35: C23.2 D4.P$2(A) IC6.4(OUT)
N$42: JP8.19 R43.1
N$43: JP8.17 R42.1
N$46: G1.+ U$5.19(VBAT)
RST: JP1.1 JP8.15 U$5.17(RESET) ; also sheet 1,2
RTCK(LPC176?_ONLY): JP8.11 R40.1 U$5.100(RTCK)
SCK: JP1.3 ; also sheet 1
TCK/SWDCLK: JP8.9 R39.2 U$5.5(TCK/SWDCLK)
TDI: JP8.5 R37.2 U$5.2(TDI)
TDO/SWO: JP8.13 R41.1 U$5.1(TDO/SWO)
TMS/SWDIO: JP8.7 R38.2 U$5.3(TMS/SWDIO)
TRST_N: JP8.3 R36.2 U$5.4(TRST)
VCC: C20.2 C22.2 IC6.3(IN) IC8.3(IN) L1.1 R26.1 X3.1 ; also sheet 4
Unconnected: G1.+@1(+) U$5.10(VDDA) U$5.11(VSSA) U$5.12(VREFP) U$5.14(RSTOUT) U$5.15(VREFN) U$5.42(VDD(REG)(3V3)1) U$5.84(VDD(REG)(3V3)2)

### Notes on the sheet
- Supply+Debug

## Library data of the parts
C1-C33 = resistor:C-EU: CAPACITOR, European symbol
D1-D4 = BAT60A:BAT60A
DMX1IN DMX1OUT DMX2IN DMX2OUT DMX3IN DMX3OUT DMX4IN DMX4OUT = con-amp:MTA03-100: AMP connector
G1 = battery:CR2032H: LI BATTERY Varta
IC6-IC8 = v-reg:LD117A?*: Low drop fixed and adjustable positive voltage regulators 1 A Source: http://www.st.com/stonline/products/literature/ds/7194/ld1117axx.pdf
IC10-IC13 = iso308x_RS485:ISO3088
JP1 = pinhead-1:PINHD-2X3: PIN HEADER
JP4 JP5 = pinhead-1:PINHD-1X3: PIN HEADER
JP6 JP7 = pinhead-1:PINHD-1X2: PIN HEADER
JP8 = pinhead-1:PINHD-2X10: PIN HEADER
JP9-JP12 = pinhead-1:PINHD-1X9: PIN HEADER
L1 = inductors:BML15H: EMIFIL (R) Chip Ferrite Bead for GHz Noise
LED1-LED8 = led:LED: LED
Q1 Q2 = crystal:CSM-7X-DU: SMD CRYSTAL; OC_FARNELL: unknown; OC_NEWARK: unknown
R1-R48 = resistor:R-EU_: RESISTOR, European symbol
S1 S2 = uwegw:TASTER_93XX: OMRON SWITCH
SELECT_USB+ SELECT_USB- = pinhead-1:PINHD-2X2: PIN HEADER
SW1 = special:SW_DIP-10: DIP SWITCH
T1 = transistor:*-PNP-: PNP Transistror
U$1 = crystal:ASE: 3.3Vdc CMOS SMD CRYSTAL CLOCK OSCILLATOR SOurce: www.abracon.com; OC_FARNELL: unknown; OC_NEWARK: unknown
U$2 = national-semiconductor:DP83848_BETTER_SYM
U$5 = lpc1xxx-v6:LPC1768/9_MULTIGATES
U$8 = linear:LM3526-L
U$9 U$10 = diodes_1:USBLC6
X1 = con-pulse:J1006F01P: PULSEJACK (TM) 1x1 Tab-UP RJ45 10/100 Base-TX RJ45 1x1 Tab-UP with LEDs 8-pin (J1 series) and 6-pin (JP series) integrated magnetics connector, designed to support applications, such as ADSL modems, LAN-on-Motherboard, and Hub and Switches. Source: www.pulseeng.com .. PulseJack-J402.pdf; OC_FARNELL: unknown; OC_NEWARK: unknown
X2 = con-yamaichi:USB-A003: USB connector; OC_FARNELL: unknown; OC_NEWARK: unknown
X3 = con-conrad:73398?: FEMALE PRINT CONNECTOR Niedervolt-Steckverbinder Distributor Conrad
X4 = con-cypressindustries:MINI-USB_4P-: MINI USB 4 Pol. Source: www.cypressindustries.com; OC_FARNELL: unknown; OC_NEWARK: unknown

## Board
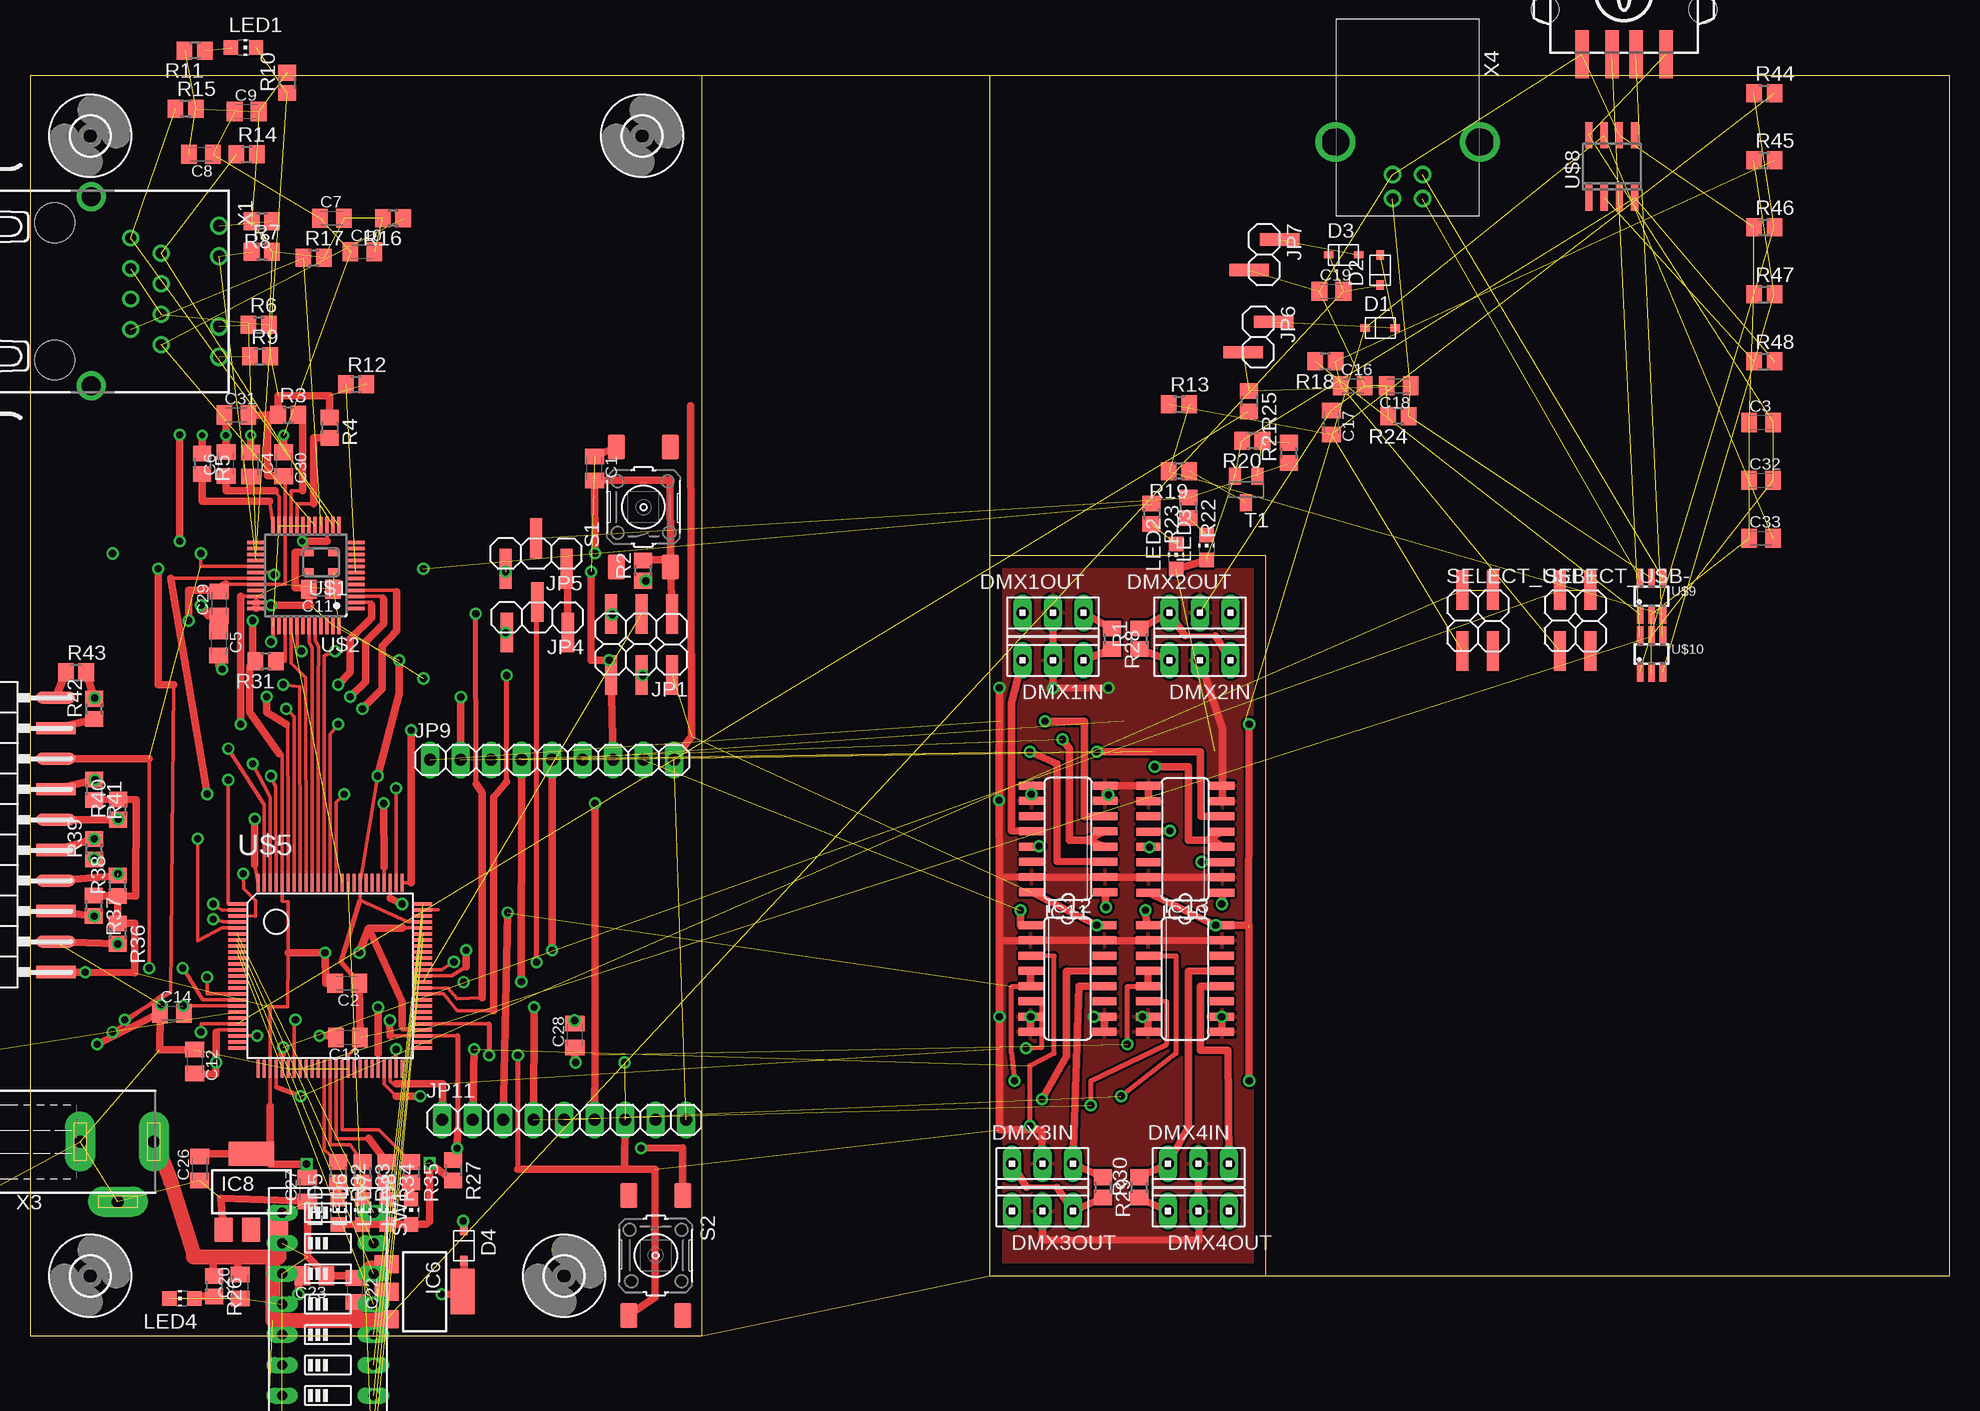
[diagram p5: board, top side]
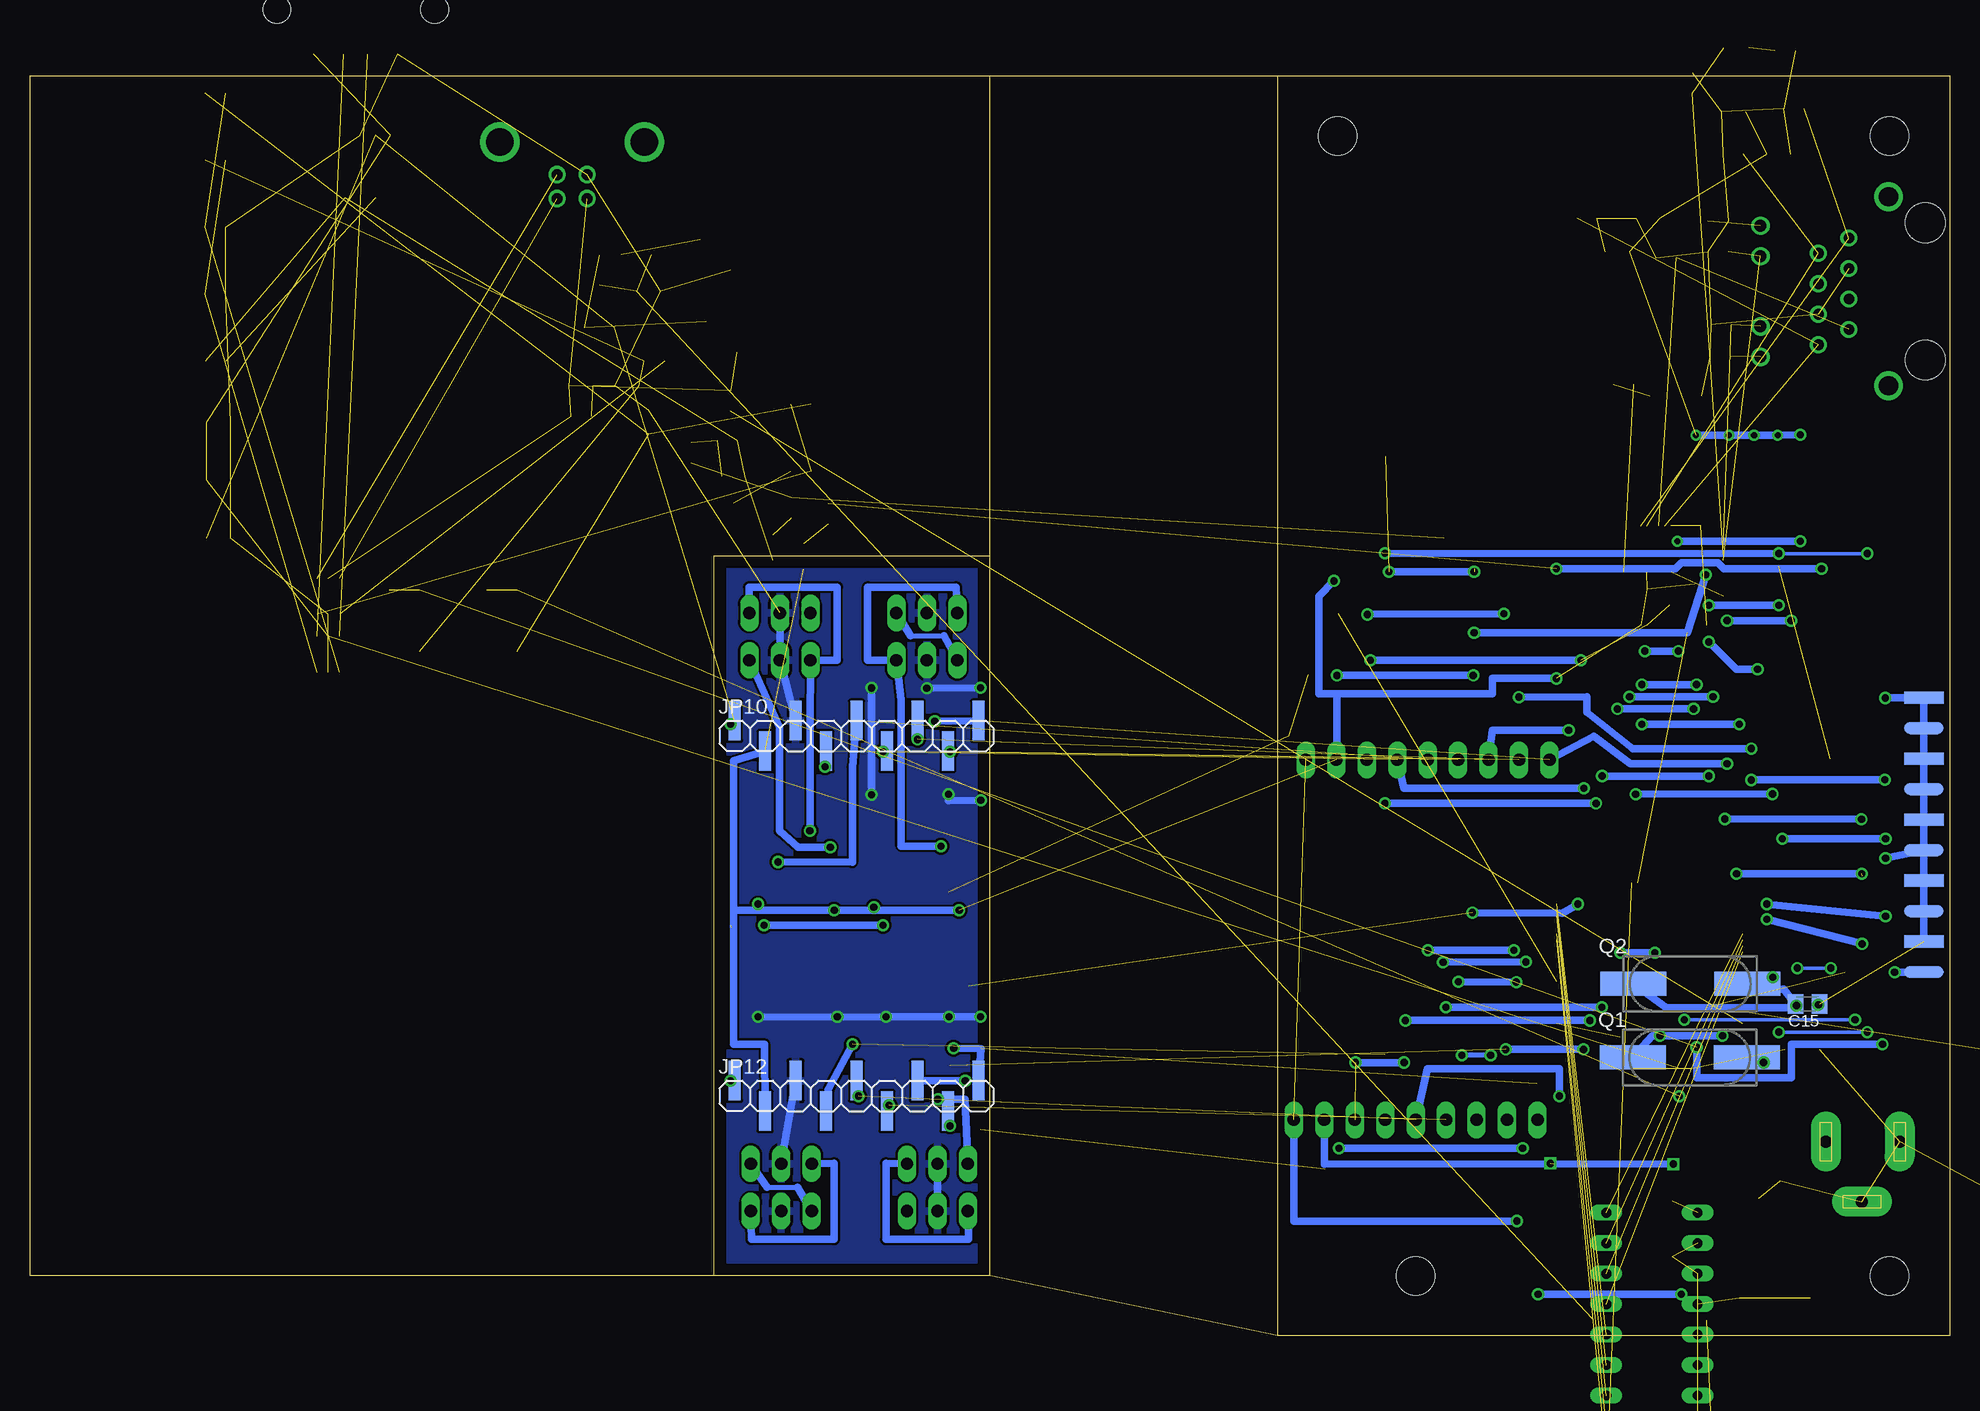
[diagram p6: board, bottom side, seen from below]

Size 160 x 105 mm. Coordinates in mm from the lower left corner, seen from the top.
Outline: 56,0 0,0 0,105 56,105
Outline: 56,0 80,5
Outline: 80,5 103,5
Outline: 103,5 160,5 160,105 80,105
Outline: 80,105 56,105
Outline: 80,5 80,65
Outline: 80,65 80,105
Outline: 56,0 56,105
Outline: 80,65 103,65 103,5
Copper layers (1*2+3*16): Top 0.035mm / dielectric 1.5mm / Route2 0.035mm / dielectric 0.15mm / Route3 0.035mm / dielectric 0.2mm / Bottom 0.035mm
Design rules "default *": minimum track width 10mil, minimum drill 24mil, track to track 8mil, track to pad 8mil, pad to pad 8mil, via to via 8mil, smd to smd 8mil, copper to edge 40mil, drill to drill 8mil, minimum pad ring 10mil, minimum via ring 8mil, stop-mask expansion 4mil, vias tented up to drill 0mil, thermal gap 10mil

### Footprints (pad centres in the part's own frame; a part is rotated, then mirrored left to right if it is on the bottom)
C0805K = smd 1.3 x 1.6: 1 -1,0; 2 1,0
BAT60A = smd 0.6 x 0.8: P$1 0,-1.25; P$2 0,1.25
10X03MTA = drill 1.016 long: 1 2.54,0; 2 0,0; 3 -2.54,0
CR2032H = drill 1.118 pad 2.54 octagon: + 5.08,10.795; +@1 -5.08,10.795; - 0,-6.985
SOT223 = smd 1.5 x 2: 1 -2.3,-3.15; 2 0,-3.15; 3 2.3,-3.15 | smd 3.8 x 2: 4 0,3.15
SO16 = smd 0.66 x 2.032: 1 -4.445,-3.073; 2 -3.175,-3.073; 3 -1.905,-3.073; 4 -0.635,-3.073; 5 0.635,-3.073; 6 1.905,-3.073; 7 3.175,-3.073; 8 4.445,-3.073; 9 4.445,3.073; 10 3.175,3.073; 11 1.905,3.073; 12 0.635,3.073; 13 -0.635,3.073; 14 -1.905,3.073; 15 -3.175,3.073; 16 -4.445,3.073
2X03SMD = smd 1.016 x 3.302: 1 -1.27,-3.81; 2 -1.27,1.27; 3 1.27,-3.81; 4 1.27,1.27; 5 3.81,-3.81; 6 3.81,1.27
1X03SMD = smd 1.016 x 3.302: 1 -1.27,1.27; 2 1.27,-1.27; 3 3.81,1.27
1X02SMD = smd 1.016 x 3.302: 1 -1.27,1.27; 2 1.27,-1.27
2X10SMD-90_2SIDES = smd 1.016 x 3.302: 1 -1.27,-3.81; 3 1.27,-3.81; 5 3.81,-3.81; 7 6.35,-3.81; 9 8.89,-3.81; 11 11.43,-3.81; 13 13.97,-3.81; 15 16.51,-3.81; 17 19.05,-3.81; 19 21.59,-3.81 | smd 1.016 x 3.302 bottom: 2 -1.27,-3.81; 4 1.27,-3.81; 6 3.81,-3.81; 8 6.35,-3.81; 10 8.89,-3.81; 12 11.43,-3.81; 14 13.97,-3.81; 16 16.51,-3.81; 18 19.05,-3.81; 20 21.59,-3.81
1X09 = drill 1.016 long: 1 -10.16,0; 2 -7.62,0; 3 -5.08,0; 4 -2.54,0; 5 0,0; 6 2.54,0; 7 5.08,0; 8 7.62,0; 9 10.16,0
1X09SMD = smd 1.016 x 3.302: 1 -1.27,1.27; 2 1.27,-1.27; 3 3.81,1.27; 4 6.35,-1.27; 5 8.89,1.27; 6 11.43,-1.27; 7 13.97,1.27; 8 16.51,-1.27; 9 19.05,1.27
0402 = smd 0.7 x 0.9: 1 -0.65,0; 2 0.65,0
CHIP-LED0805 = smd 1.2 x 1.2: A 0,-1.05; C 0,1.05
CSM-7X-DU = smd 5.5 x 2: 1 -4.75,0; 2 4.75,0
R0805 = smd 1.3 x 1.5: 1 -0.85,0; 2 0.85,0
TASTER_93XX = smd 2.1 x 1.4: 1 -5,2.25; 2 5,2.25; 3 -5,-2.25; 4 5,-2.25
2X02SMD = smd 1.016 x 3.302: 1 -1.27,-3.81; 2 -1.27,1.27; 3 1.27,-3.81; 4 1.27,1.27
EDG-10 = drill 0.813 long: 1 -11.43,-3.81; 2 -8.89,-3.81; 3 -6.35,-3.81; 4 -3.81,-3.81; 5 -1.27,-3.81; 6 1.27,-3.81; 7 3.81,-3.81; 8 6.35,-3.81; 9 8.89,-3.81; 10 11.43,-3.81; 11 11.43,3.81; 12 8.89,3.81; 13 6.35,3.81; 14 3.81,3.81; 15 1.27,3.81; 16 -1.27,3.81; 17 -3.81,3.81; 18 -6.35,3.81; 19 -8.89,3.81; 20 -11.43,3.81
SOT23-BEC = smd 1 x 1.4: B -0.95,-1.1; C 0,1.1; E 0.95,-1.1
ASE = smd 0.9 x 0.65: 1 -1.05,-0.825; 2 1.05,-0.825; 3 1.05,0.825; 4 -1.05,0.825
LQFP48 = smd 1.5 x 0.3: 1 -4.15,2.75; 2 -4.15,2.25; 3 -4.15,1.75; 4 -4.15,1.25; 5 -4.15,0.75; 6 -4.15,0.25; 7 -4.15,-0.25; 8 -4.15,-0.75; 9 -4.15,-1.25; 10 -4.15,-1.75; 11 -4.15,-2.25; 12 -4.15,-2.75; 25 4.15,-2.75; 26 4.15,-2.25; 27 4.15,-1.75; 28 4.15,-1.25; 29 4.15,-0.75; 30 4.15,-0.25; 31 4.15,0.25; 32 4.15,0.75; 33 4.15,1.25; 34 4.15,1.75; 35 4.15,2.25; 36 4.15,2.75 | smd 0.3 x 1.5: 13 -2.75,-4.15; 14 -2.25,-4.15; 15 -1.75,-4.15; 16 -1.25,-4.15; 17 -0.75,-4.15; 18 -0.25,-4.15; 19 0.25,-4.15; 20 0.75,-4.15; 21 1.25,-4.15; 22 1.75,-4.15; 23 2.25,-4.15; 24 2.75,-4.15; 37 2.75,4.15; 38 2.25,4.15; 39 1.75,4.15; 40 1.25,4.15; 41 0.75,4.15; 42 0.25,4.15; 43 -0.25,4.15; 44 -0.75,4.15; 45 -1.25,4.15; 46 -1.75,4.15; 47 -2.25,4.15; 48 -2.75,4.15
3,2 = hole 3.2: 0,0
LQFP100-14X14 = smd 0.27 x 1.5: 1 -6,-7.75; 2 -5.5,-7.75; 3 -5,-7.75; 4 -4.5,-7.75; 5 -4,-7.75; 6 -3.5,-7.75; 7 -3,-7.75; 8 -2.5,-7.75; 9 -2,-7.75; 10 -1.5,-7.75; 11 -1,-7.75; 12 -0.5,-7.75; 13 0,-7.75; 14 0.5,-7.75; 15 1,-7.75; 16 1.5,-7.75; 17 2,-7.75; 18 2.5,-7.75; 19 3,-7.75; 20 3.5,-7.75; 21 4,-7.75; 22 4.5,-7.75; 23 5,-7.75; 24 5.5,-7.75; 25 6,-7.75; 51 6,7.75; 52 5.5,7.75; 53 5,7.75; 54 4.5,7.75; 55 4,7.75; 56 3.5,7.75; 57 3,7.75; 58 2.5,7.75; 59 2,7.75; 60 1.5,7.75; 61 1,7.75; 62 0.5,7.75; 63 0,7.75; 64 -0.5,7.75; 65 -1,7.75; 66 -1.5,7.75; 67 -2,7.75; 68 -2.5,7.75; 69 -3,7.75; 70 -3.5,7.75; 71 -4,7.75; 72 -4.5,7.75; 73 -5,7.75; 74 -5.5,7.75; 75 -6,7.75 | smd 1.5 x 0.27: 26 7.75,-6; 27 7.75,-5.5; 28 7.75,-5; 29 7.75,-4.5; 30 7.75,-4; 31 7.75,-3.5; 32 7.75,-3; 33 7.75,-2.5; 34 7.75,-2; 35 7.75,-1.5; 36 7.75,-1; 37 7.75,-0.5; 38 7.75,0; 39 7.75,0.5; 40 7.75,1; 41 7.75,1.5; 42 7.75,2; 43 7.75,2.5; 44 7.75,3; 45 7.75,3.5; 46 7.75,4; 47 7.75,4.5; 48 7.75,5; 49 7.75,5.5; 50 7.75,6; 76 -7.75,6; 77 -7.75,5.5; 78 -7.75,5; 79 -7.75,4.5; 80 -7.75,4; 81 -7.75,3.5; 82 -7.75,3; 83 -7.75,2.5; 84 -7.75,2; 85 -7.75,1.5; 86 -7.75,1; 87 -7.75,0.5; 88 -7.75,0; 89 -7.75,-0.5; 90 -7.75,-1; 91 -7.75,-1.5; 92 -7.75,-2; 93 -7.75,-2.5; 94 -7.75,-3; 95 -7.75,-3.5; 96 -7.75,-4; 97 -7.75,-4.5; 98 -7.75,-5; 99 -7.75,-5.5; 100 -7.75,-6
SO08 = smd 0.6 x 2.2: 1 -1.905,-2.6; 2 -0.635,-2.6; 3 0.635,-2.6; 4 1.905,-2.6; 5 1.905,2.6; 6 0.635,2.6; 7 -0.635,2.6; 8 -1.905,2.6
SOT23-6 = smd 0.55 x 1.6: 1 -0.95,-1.5; 2 0,-1.5; 3 0.95,-1.5; 4 0.95,1.5; 5 0,1.5; 6 -0.95,1.5
J1 = drill 0.9 pad 1.3: 1 4.445,2.54; 2 3.175,0; 3 1.905,2.54; 4 0.635,0; 5 -0.635,2.54; 6 -1.905,0; 7 -3.175,2.54; 8 -4.445,0 | drill 1 pad 1.422: 9 5.465,7.37; 10 2.925,7.37; 11 -2.925,7.37; 12 -5.465,7.37 | drill 1.6 pad 2.184: M1 -7.875,-3.3; M2 7.875,-3.3 | hole 3.3: 5.715,-6.35; -5.715,-6.35
USB-A003 = smd 1.12 x 4: 1 -3.5,14; 2 -1,14; 3 1,14; 4 3.5,14 | hole 2.3: -6.57,10.28; 6.57,10.28
733980-62 = drill 1 pad 2.5 long: 1 0,8.57; 2 0,2.42; 3 5,5.57
85-32004-10X = drill 0.92 pad 1.27: 1 4.71,-1.25; 2 4.71,1.25; 3 2.71,1.25; 4 2.71,-1.25 | drill 2.3 pad 3: M1 0,6.02; M2 0,-6.02

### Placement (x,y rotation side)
C1  47.03,72.29 270 top
C2  26.42,29.38 180 top
C3  144.27,76.12 0 top
C4  18.37,72.63 270 top
C5  15.72,57.71 270 top
C6  16.32,72.67 90 top
C7  25.15,93.14 0 top
C8  14.22,98.47 180 top
C9  18.03,102.03 0 top
C10  27.69,90.34 0 top
C11  24.23,62.23 180 top
C12  13.72,22.86 270 top
C13  26.48,24.87 180 top
C14  11.82,26.89 0 top
C15  11.84,27.66 180 bottom
C16  110.24,79.17 0 top
C17  108.46,76.12 270 top
C18  114.05,79.17 180 top
C19  108.46,87.04 0 top
C20  17.51,4.13 90 top
C21  not placed on the board
C22  27.07,3.82 270 top
C23  23.67,5.02 180 top
C24  not placed on the board
C25  not placed on the board
C26  14.12,13.94 90 top
C27  23.1,12.21 90 top
C28  45.38,25.04 90 top
C29  15.74,61.03 90 top
C30  21.13,72.64 270 top
C31  17.17,76.74 0 top
C32  144.27,71.29 0 top
C33  144.27,66.47 0 top
D1  112.52,83.99 270 top
D2  112.52,88.82 0 top
D3  109.47,90.09 270 top
D4  36.14,7.53 180 top
DMX1IN  85.25,56.3 0 top
DMX1OUT  85.25,60.25 180 top
DMX2IN  97.5,56.3 0 top
DMX2OUT  97.5,60.25 180 top
DMX3IN  84.37,14.35 180 top
DMX3OUT  84.37,10.4 0 top
DMX4IN  97.38,14.35 180 top
DMX4OUT  97.38,10.4 0 top
G1  not placed on the board
IC6  32.87,3.68 270 top
IC7  not placed on the board
IC8  18.43,12.01 0 top
IC10  96.28,41.39 90 top
IC11  86.51,41.41 90 top
IC12  86.46,29.78 270 top
IC13  96.25,29.78 270 top
JP1  52.22,56.36 180 top
JP4  43.53,59.88 180 top
JP5  43.43,65.2 180 top
JP6  102.36,83.23 270 top
JP7  102.87,90.09 270 top
JP8  -1.68,31.59 90 top
JP9  43.5,48 0 top
JP10  100,50 0 bottom
JP11  44.5,18 0 top
JP12  100,20 0 bottom
L1  not placed on the board
LED1  17.78,107.36 270 top
LED2  95.5,64.94 0 top
LED3  98.04,65.71 0 top
LED4  12.63,3.13 90 top
LED5  25.65,10.33 0 top
LED6  27.69,10.33 0 top
LED7  29.72,10.33 0 top
LED8  31.75,10.33 0 top
Q1  21.67,23.2 0 bottom
Q2  21.61,29.33 0 bottom
R1  92.46,58.09 90 top
R2  51.09,63.78 90 top
R3  21.51,76.75 0 top
R4  24.97,75.69 270 top
R5  14.35,72.69 270 top
R6  19.05,84.25 0 top
R7  19.3,90.34 0 top
R8  19.3,92.88 180 top
R9  19.15,81.62 0 top
R10  21.43,104.41 90 top
R11  13.72,107.11 180 top
R12  27.16,79.29 0 top
R13  95.76,77.64 0 top
R14  18.03,98.47 0 top
R15  12.95,102.28 0 top
R16  30.23,93.14 180 top
R17  23.62,89.84 0 top
R18  107.95,81.2 180 top
R19  95.76,72.06 180 top
R20  101.85,74.6 180 top
R21  104.9,73.58 90 top
R22  96.52,69.01 270 top
R23  93.47,68.5 270 top
R24  114.05,76.63 180 top
R25  101.6,77.9 270 top
R26  15.34,4.14 270 top
R27  35.26,13.8 270 top
R28  90.17,58.09 270 top
R29  89.41,12.37 270 top
R30  92.46,12.37 90 top
R31  19.62,56.23 180 top
R32  25.65,13.64 270 top
R33  27.69,13.64 270 top
R34  29.72,13.64 270 top
R35  31.75,13.64 270 top
R36  7.29,33.52 270 top
R37  5.28,35.84 270 top
R38  7.29,37.51 90 top
R39  5.33,40.56 90 top
R40  7.32,43.86 90 top
R41  5.33,45.51 270 top
R42  5.33,52.24 90 top
R43  3.81,55.29 0 top
R44  144.53,103.55 0 top
R45  144.53,97.96 0 top
R46  144.53,92.38 0 top
R47  144.53,86.79 0 top
R48  144.53,81.2 0 top
S1  51.11,69.07 90 top
S2  52.13,6.7 270 top
SELECT_USB+  120.65,60.88 0 top
SELECT_USB-  128.78,60.88 0 top
SW1  24.8,-1.16 270 top
T1  101.35,70.53 180 top
U$1  24.23,64.47 180 top
U$2  22.99,63.38 180 top
U$3  [3,2]  5,5 0 top
U$4  [3,2]  44.5,5 0 top
U$5  25,30 270 top
U$6  [3,2]  5,100 0 top
U$7  [3,2]  51,100 0 top
U$8  131.83,97.46 0 top
U$9  135.13,61.64 0 top
U$10  135.13,56.82 0 top
X1  8.38,87.04 270 top
X2  132.84,120.82 180 top
X3  1.74,16.18 270 top
X4  114.81,99.49 270 top

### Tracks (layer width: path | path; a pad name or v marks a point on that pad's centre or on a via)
+3.3VA  (2 unrouted)
+3V3  (via drill 0.6)  (29 unrouted)
  Top 0.305: 21.23,71.61 U$2.22 21.24,62.63 U$2.32 16.35,62.63 | 20,19.16 U$5.28 20,27.42 21.46,27.43 21.48,31.94 21.49,36.19 21.01,36.22 U$5.96 21.01,48.46 20.75,48.52 | U$5.71 31.03,34 | U$5.54 30.99,25.5 30.99,25.83
  Top 0.61: 21.23,71.61 21.13,71.61 C30.2 21.13,71.66 19.78,71.66 19.78,76.75 R3.1 | R3.1 C31.2 | R3.1 20.68,76.74 20.68,78.36 24.97,78.36 R4.1 | 19.99,14.32 IC8.4 14.12,15.16 C26.2 | 19.99,14.32 v23.02,14.32 C27.2 | 20,19.16 19.99,14.32 | 20.75,48.52 18.29,51.99 18.29,55.75 R31.2 18.54,56.71 v18.54,59.61 | v13.21,59.61 13.21,62.15 15.62,62.15 arc-90 C29.2 arc-90 16.35,62.63 | 31.03,34 30.99,33.96 28.19,33.96 | 28.19,33.96 v27.43,31.92 | 30.99,25.83 30.99,27.86 28.19,33.96 | LED5.A LED6.A LED7.A LED8.A 32.99,9.28 33.27,9.57 v33.27,14.37 R27.2 | IC13.1 92.93,35.23 v92.96,35.48 | v82.55,35.48 82.55,34.22 IC12.1 | C2.2 24.64,29.38 v24.56,31.92 21.48,31.94 | LED2.A LED3.A | v51.31,62.91 51.31,62.93 R2.1 | IC11.1 v89.66,35.71 | IC10.1 v99.31,35.99 | R41.2 R40.2 8.81,44.67 8.79,36.62 R38.1 | R38.1 R37.1 | R38.1 R36.1 8.71,34.39 8.71,30.27 v4.58,30.3 JP8.1
  Bottom 0.61: v18.54,59.61 v13.21,59.61 | v27.43,31.92 v24.56,31.92 | v23.02,14.32 32.97,14.35 52.12,14.32 52.12,17.62 JP11.8 | 89.66,35.48 v92.96,35.48 arc-90 93.22,35.48 99.31,35.48 | 89.66,35.48 v82.55,35.48 | 101.35,35.48 101.35,24.3 98.78,24.3 JP12.2 | 101.35,35.48 101.35,47.93 JP10.2 | 99.31,35.48 101.35,35.48 | v32.77,54.78 38.1,54.78 38.1,53.51 51.05,53.51 | 51.05,53.51 51.05,50 JP9.8 | 51.05,53.51 52.58,53.51 52.58,61.64 v51.31,62.91 | v89.66,35.71 89.66,35.48 | v99.31,35.99 99.31,35.48 | JP8.1 v4.58,30.3
+5V  (via drill 0.6)  (7 unrouted)
  Top 0.61: 101.55,34.06 101.6,45.64 v101.6,50.97 | IC12.16 89.41,34.22 v88.9,34.21 IC11.16 | v36.07,9.57 D4.P$1 | JP9.9 55.12,49.96 55.04,77.52 | v101.6,21.26 101.59,34.22 IC13.16 99.07,34.21 v98.81,34.21 IC10.16
  Bottom 0.61: v98.81,34.21 v88.9,34.21 | JP11.9 54.66,9.57 v36.07,9.57 | JP10.1 101.35,51.23 v101.6,50.97 | v101.6,21.26 JP12.1
BUTTON_RESERVE  (via drill 0.6)
  Top 0.305: 30,25.02 U$5.53 35.61,25.02
  Top 0.406: 35.61,25.02 35.61,17.19
  Top 0.61: 30,25.02 29.97,26.08 v29.97,26.29 | v45.36,26.29 C28.2 | R27.1 v35.59,15.64 35.61,17.19 | v50.9,15.64 54.36,15.67 S2.1
  Bottom 0.61: v29.97,26.29 v45.36,26.29 | v35.59,15.64 41.1,15.62 v50.9,15.64
D+  (via drill 0.6)  (2 unrouted)
  Top 0.305: 20.5,20.72 U$5.29
  Top 0.406: v22.53,19.96 20.5,20.72
D-  (via drill 0.6)  (2 unrouted)
  Top 0.305: U$5.30 21,23.46
  Top 0.61: 21,23.46 v21.08,24.05 | v5.59,24.3 10.16,26.59
  Bottom 0.61: v5.59,24.3 13.21,24.3 13.21,21.51 21.08,21.51 v21.08,24.05
DERE0  (via drill 0.6)  (1 unrouted)
  Top 0.305: U$5.76 31.73,37.75
  Top 0.61: 31.73,37.75 v31.75,50.47 | v86.03,49.7 86.61,48.94 86.61,41.32 88.14,41.32 | 88.14,41.32 IC11.4 | IC11.5 88.14,41.32
  Bottom 0.61: v31.75,50.47 38.1,50.47 JP9.3 | JP10.7 v86.03,49.7
DERE1  (via drill 0.6)  (1 unrouted)
  Top 0.305: U$5.77 30.5,38 v30.48,45.64
  Top 0.61: v93.73,47.42 96.52,47.42 96.52,41.32 98.04,41.32 98.33,41.48 | 98.33,41.48 IC10.5 | IC10.4 98.33,41.48
  Bottom 0.61: v30.48,45.64 45.47,45.64 JP9.6 | JP10.4 v93.73,47.42
DERE2  (via drill 0.6)  (1 unrouted)
  Top 0.305: U$5.78 30,36.47
  Top 0.406: IC12.5 81.79,29.13 81.79,23.54 v82.04,21.26
  Top 0.61: 30,36.47 v30.99,35.99 | IC12.5 IC12.4 | v39.78,35.28 JP11.3
  Bottom 0.61: v30.99,35.99 32.26,35.23 v39.78,35.28 | v82.04,21.26 85.85,21.26 JP12.7
DERE3  (via drill 0.6)  (1 unrouted)
  Top 0.305: U$5.79 29.5,39.07
  Top 0.406: v91.44,24.3 91.44,29.13 IC13.5
  Top 0.61: 29.5,39.07 v29.46,44.37 | v47.07,44.37 47.07,23.44 JP11.6 | IC13.4 IC13.5
  Bottom 0.61: v29.46,44.37 v47.07,44.37 | v91.44,24.3 93.47,20.49 JP12.4
DIP1_DMX1_IN/OUT  (1 unrouted)
DIP2_DMX2_IN/OUT  (1 unrouted)
DIP3_DMX3_IN/OUT  (1 unrouted)
DIP4_DMX4_IN/OUT  (1 unrouted)
DIP5  (1 unrouted)
DIP6  (1 unrouted)
  Top 0.305: 34.02,35.5 U$5.74
DIP7  (1 unrouted)
DIP8  (1 unrouted)
DIP9  (1 unrouted)
DIP10_NETMASK  (1 unrouted)
ENET_CRS
  Top 0.305: U$5.92 22.96,54.84 21.74,56.06 U$2.40
ENET_MDC  (via drill 0.6)
  Top 0.305: U$2.31 11.68,63.13 | v26.16,45.13 25.5,44.47 U$5.87
  Top 0.61: 11.68,63.13 v14.76,45.16
  Bottom 0.61: v14.76,45.16 v26.16,45.13
ENET_MDIO  (via drill 0.6)  (1 unrouted)
  Top 0.305: v20.32,63.42 20.18,63.62 U$2.30
  Top 0.61: JP4.3 39.62,58.61 v39.62,58.59
  Bottom 0.61: v39.62,58.59 21.84,58.59 v20.32,63.42
ENET_MDIO/USB  (via drill 0.6)
  Top 0.305: U$5.64 34.29,30.5 v35.31,31.16
  Top 0.406: v42.22,31.14 42.22,60.35
  Top 0.61: 42.22,60.35 42.26,60.35 JP4.2
  Bottom 0.61: v35.31,31.16 v42.22,31.14
ENET_REF_CLK  (via drill 0.6)  (1 unrouted)
  Top 0.305: U$5.88 25,50.14 v25.65,50.97 | 17.53,61.63 U$2.34
  Top 0.61: v17.53,50.97 17.53,61.63
  Bottom 0.61: v25.65,50.97 v17.53,50.97
ENET_RX_ER  (via drill 0.6)
  Top 0.305: U$2.41 22.24,57.44 v22.61,57.07 | v25.4,57.07 24.51,56.69 24.51,37.81 U$5.89
  Bottom 0.61: v22.61,57.07 v25.4,57.07
ENET_RXD0
  Top 0.305: U$5.91 23.5,37.85 23.5,55.16 23.49,56.19 23.5,57.32 23.24,57.86 U$2.43
ENET_RXD1
  Top 0.305: U$2.44 23.74,57.97 24.03,57.43 24.03,56.44 24,55.24 24,37.8 U$5.90
ENET_TX_EN  (via drill 0.6)
  Top 0.305: U$5.93 22.45,54.1 v21.08,54.28 | 28.45,60.88 28.45,61.13 U$2.2
  Top 0.61: v25.65,54.28 26.67,55.29 26.67,58.09 28.45,59.86 28.45,60.88
  Bottom 0.61: v21.08,54.28 v25.65,54.28
ENET_TXD0  (via drill 0.6)
  Top 0.305: U$2.3 27.14,61.64 29.46,61.64 29.46,61.39 | 21.34,50.97 21.46,51 21.49,42.31 21.49,37.84 U$5.95
  Top 0.61: 29.46,61.39 29.46,59.36 27.94,57.83 27.94,54.53 v26.67,53.26 | v19.71,53.26 19.71,51.99 21.34,50.97
  Bottom 0.61: v26.67,53.26 v19.71,53.26
ENET_TXD1  (via drill 0.6)
  Top 0.305: U$5.94 22,51.58 v21.34,52.24 | 30.56,62.02 30.56,62.13 U$2.4
  Top 0.61: v27.69,52.24 27.94,52.55 29.31,53.92 29.31,57.48 30.56,58.75 30.56,62.02
  Bottom 0.61: v21.34,52.24 v27.69,52.24
GND  (via drill 0.5, 0.6)  (51 unrouted)
  Top 0.305: U$2.15 24.76,66.21 | v22.68,66.21 U$2.19 | U$2.35 19.81,61.13 arc-90 v20.07,60.88 | U$5.55 38.24,26 | U$5.41 26.5,23.37 27.43,24.3 27.43,24.82 C13.1 | U$5.72 31.45,34.52 27.51,36.29 U$5.83 v28.96,46.66 | U$5.97 20.47,45.72 v20.07,46.66
  Top 0.406: C2.1 25.91,31.16 27.51,36.29 | 38.24,26 v38.25,23.39 | v40.64,23.39 40.64,13.89
  Top 0.61: C4.1 v18.37,75.06 v18.38,75.06 | v21.13,75.06 C30.1 | R5.1 14.35,75.06 v14.33,75.06 | C6.2 v16.32,75.06 v16.28,75.06 | v16.33,75.06 16.33,76.74 C31.1 | IC8.1 15.88,11.47 C27.1 23.1,6.58 C23.1 26.87,5.02 C22.1 28.23,5.98 IC6.1 | C5.1 arc90 15.74,58.74 C29.1 14.82,60.03 v14.22,60.88 | U$2.36 U$2.35 | C28.1 v45.47,22.78 | v80.77,54.02 v80.75,44.62 80.77,38.27 | 80.77,38.27 80.77,32.94 | 80.77,32.94 v80.77,26.59 80.77,17.19 84.33,17.19 DMX3IN.2 | IC12.9 IC12.10 v88.65,26.59 | IC13.8 IC13.7 92.71,26.6 v92.71,26.59 | IC13.10 IC13.9 v99.31,26.59 | IC12.8 IC12.7 v83.39,26.59 | IC13.15 99.82,32.95 99.82,32.94 IC13.2 92.93,32.94 89.28,32.94 IC12.15 IC12.2 | C2.1 C13.1 | C12.1 10.79,23.85 C14.1 v10.92,27.61 | JP9.7 JP1.6 v48.26,56.31 46.74,56.31 v46.74,63.67 | S1.2 C1.1 | v28.96,46.66 30.73,53.51 v30.73,56.31 | v12.45,66.21 v12.45,75.1 | 24.76,66.21 v22.68,66.21 U$1.2 22.07,65.3 22.07,62.35 23.23,62.35 C11.2 23.23,60.88 | v20.07,60.88 23.23,60.88 | 23.37,60.88 23.23,60.88 | DMX3OUT.2 84.35,8.02 97.41,7.97 DMX4OUT.2 DMX4IN.2 | 99.57,38.27 IC10.2 IC10.15 IC11.2 IC11.15 80.77,38.27 | 80.77,32.94 83.31,32.94 | IC11.10 v83.44,45.13 IC11.9 | IC10.7 IC10.8 99.36,50.64 DMX2IN.2 | IC10.10 IC10.9 IC11.8 | IC11.8 IC11.7 | IC11.8 v89.86,45.11 | v89.86,54 v85.24,53.97 DMX1IN.2 DMX1OUT.2 | 40.64,13.89 49.53,13.89 | 49.53,13.89 JP11.7 | 49.53,13.89 52.07,13.89 52.07,3.22 S2.4 | R39.1 v5.33,39.8 | R43.2 R42.2 v5.36,53.16
  Bottom 0.406: v38.25,23.39 v40.64,23.39
  Bottom 0.61: v21.13,75.06 v18.38,75.06 v16.33,75.06 v16.28,75.06 v14.33,75.06 v12.45,75.1 | v20.07,60.88 v14.22,60.88 | JP8.10 JP8.12 JP8.14 JP8.16 JP8.18 JP8.20 v5.36,53.16 | JP8.10 JP8.8 JP8.6 JP8.4 | v45.47,22.78 v49.53,22.78 | v99.31,26.59 92.61,26.54 | 92.61,26.54 v88.65,26.59 v83.39,26.59 v80.77,26.59 | v92.71,26.59 92.86,26.59 92.61,26.54 | v20.07,46.66 v28.96,46.66 | C15.1 v10.92,27.61 | v30.73,56.31 v48.26,56.31 | v22.68,66.21 v12.45,66.21 | v39.62,63.67 v46.74,63.67 | DMX3IN.2 DMX3OUT.2 | DMX4IN.2 JP12.3 | IC11.10 v80.75,44.62 | JP10.3 DMX2IN.2 DMX2OUT.2 | v80.77,54.02 v85.24,53.97 | v89.86,45.11 v89.86,54 | v5.33,39.8 JP8.10
  pour Bottom: 102.85,5.14 80.01,5 79.86,65.07 103,65.06
  pour Top: 79.86,5.19 80.01,64.69 102.89,64.93 103.08,4.9
LED_ACT  (2 unrouted)
LED_DMX1_RECEIV_DATA
  Top 0.305: U$5.37 24.5,15.5 R32.1
LED_DMX2_RECEIV_DATA
  Top 0.305: U$5.38 25,15.92 26.67,15.92 R33.1
LED_DMX3_RECEIV_DATA
  Top 0.305: U$5.39 25.5,16.43 28.19,16.43 28.19,16.45
  Top 0.61: 28.19,16.45 R34.1
LED_DMX4_RECEIV_DATA
  Top 0.305: U$5.40 26,17.19 29.04,17.19 R35.1
LED_LINK  (2 unrouted)
LED_SPEED  (2 unrouted)
MISO  (via drill 0.6)
  Top 0.305: U$5.61 34.82,28.98 35.56,28.11 37.64,28.16
  Top 0.406: 37.16,46.02 37.14,60.12
  Top 0.61: 37.64,28.16 37.67,45.26 37.16,46.02 | JP1.5 v48.51,60.12 | v37.13,60.17 37.14,60.12
  Bottom 0.61: v48.51,60.12 v37.13,60.17
MOSI  (via drill 0.6)
  Top 0.305: U$5.60 34.44,28.5 35.56,27.1 38.61,27.1 | JP1.4 v51.05,55.04
  Top 0.406: 39.7,46.17 v39.7,55.04
  Top 0.61: 38.61,27.1 38.61,44.88 39.7,46.17
  Bottom 0.61: v39.7,55.04 v51.05,55.04
N$1  (via drill 0.6)
  Top 0.61: v95,42.08 IC10.12 | R1.1 DMX2IN.3
  Bottom 0.61: v95,42.08 95,50.72 DMX2IN.3 92.71,56.31 92.71,62.4 100.08,62.4 DMX2OUT.3
N$2  (via drill 0.6)
  Top 0.406: 96.27,58.34 98.81,58.34
  Top 0.61: v93.29,40.71 IC10.13 | R1.2 DMX2OUT.1 96.27,58.34 | 98.81,58.34 DMX2IN.1
  Bottom 0.61: DMX2IN.1 97.54,50.72 97.54,42.08 95.96,40.74 v93.29,40.71
N$4  (1 unrouted)
N$5
  Top 0.61: R32.2 LED5.C
N$6
  Top 0.61: R33.2 LED6.C
N$8  (1 unrouted)
N$9  (1 unrouted)
N$10  (1 unrouted)
N$11  (2 unrouted)
N$12  (via drill 0.6)
  Top 0.305: 15.49,25.32 15.67,25.5 U$5.22
  Top 0.61: 15.49,25.32 v15.49,22.78 15.47,21.82 C12.2
  Bottom 0.61: Q1.2 15.49,23.28 v15.49,22.78
N$13  (via drill 0.6)
  Top 0.305: v18.92,25.02 18.91,25 U$5.23
  Top 0.61: C13.2 25.33,25.02 v24.13,25.02
  Bottom 0.61: Q1.1 24.78,25.02 v24.13,25.02 v18.92,25.02
N$14
  Top 0.305: U$2.21 21.73,70.41 22.71,70.41
  Top 0.61: 22.71,70.41 22.68,76.75 R3.2
N$15
  Top 0.305: 23.64,69.35 22.23,69.35 U$2.20
  Top 0.61: R4.2 23.64,74.84 23.64,69.35
N$16  (via drill 0.6)
  Top 0.305: U$5.18 14.74,27.5 14.73,27.5 v12.76,27.52
  Top 0.61: v12.76,27.52 C14.2
  Bottom 0.61: Q2.1 23.62,27.35 12.95,27.35 v12.76,27.52
N$17  (via drill 0.6)  (2 unrouted)
  Top 0.305: U$2.23 20.75,69.92 20.43,70.41 | 20.24,58 U$2.37
  Top 0.61: 20.43,70.41 18.38,70.41 | 18.38,70.41 C4.2 | C6.1 16.32,70.41 18.38,70.41 | C5.2 15.72,55.83 v16,55.55 | v20.07,57.83 20.24,58
  Bottom 0.61: v16,55.55 17.78,55.55 v20.07,57.83
N$18
  Top 0.305: U$2.24 19.94,69.57
  Top 0.61: 19.94,69.57 14.31,69.55 14.33,71.11 14.33,71.82 R5.2
N$19
  Top 0.305: U$2.39 21.24,56.23 R31.1
N$20  (via drill 0.6)
  Top 0.305: v14.73,29.89 14.73,28.52 14.75,28.5 U$5.16
  Bottom 0.61: Q2.2 15.01,28.9 | 15.01,28.9 14.73,29.18 v14.73,29.89 | C15.2 13.83,28.9 15.01,28.9
N$21  (1 unrouted)
N$22  (1 unrouted)
N$23  (2 unrouted)
N$24  (2 unrouted)
N$25  (2 unrouted)
N$26  (1 unrouted)
N$27  (1 unrouted)
N$28  (2 unrouted)
N$29  (1 unrouted)
N$30  (5 unrouted)
N$31  (2 unrouted)
N$32
  Top 0.61: R26.2 13.68,3.29 LED4.A
N$33  (1 unrouted)
N$34  (1 unrouted)
N$35  (via drill 0.6)
  Top 0.61: C23.2 22.35,4.7 v22.35,3.48 | v34.29,3.48 35.82,3.48 arc90 IC6.4 36.11,3.68 D4.P$2
  Bottom 0.61: v22.35,3.48 v34.29,3.48
N$36
  Top 0.61: IC11.12 81.79,42.08 81.79,52.75 DMX1IN.3 | DMX1OUT.3 R28.1
  Bottom 0.406: 86.61,58.34 83.82,58.34
  Bottom 0.61: DMX1OUT.3 86.61,58.34 | 83.82,58.34 DMX1IN.3
N$37  (via drill 0.6)
  Top 0.61: IC11.13 v84.07,40.81 | R28.2 DMX1IN.1
  Bottom 0.61: v84.07,40.81 87.38,40.81 87.38,53.01 DMX1IN.1 90.17,56.31 90.17,62.4 82.8,62.4 DMX1OUT.1
N$38
  Top 0.61: IC12.12 87.4,29.13 DMX3IN.3 R29.1
  Bottom 0.61: DMX3IN.3 88.65,14.4 88.65,8.05 81.79,8.05 DMX3OUT.3
N$39  (via drill 0.6)
  Top 0.406: 85.6,12.37 83.06,12.37
  Top 0.61: R29.2 DMX3OUT.1 85.6,12.37 | 83.06,12.37 DMX3IN.1 | v84.33,19.73 86.36,23.29 86.36,30.4 IC12.13
  Bottom 0.61: DMX3IN.1 82.04,19.73 v84.33,19.73
N$40
  Top 0.61: DMX4IN.3 99.82,23.8 97.54,23.8 97.54,29.13 IC13.12 | DMX4OUT.3 R30.1
  Bottom 0.406: 98.55,12.37 96.01,12.37
  Bottom 0.61: DMX4IN.3 98.55,12.37 | 96.01,12.37 DMX4OUT.3
N$41
  Top 0.61: IC13.13 96.52,30.4 96.52,17.45 DMX4IN.1 R30.2
  Bottom 0.61: DMX4IN.1 92.96,14.4 92.96,8.05 99.87,8.05 DMX4OUT.1
N$42
  Top 0.61: R43.1 JP8.19
N$43
  Top 0.61: R42.1 JP8.17
N$44
  Top 0.61: R34.2 LED7.C
N$45
  Top 0.61: R35.2 LED8.C
N$46  (1 unrouted)
N$47  (1 unrouted)
N$48  (1 unrouted)
RD+  (2 unrouted)
RD-  (2 unrouted)
RST  (via drill 0.6)  (1 unrouted)
  Top 0.305: U$2.29 14.22,64.13 v14.22,65.2 | 9.93,48.1 v9.91,30.65 | v12.7,30.65 12.72,30.65 14.35,28.01 17.24,28.01 U$5.17
  Top 0.61: JP1.1 S1.3 53.36,64.69 | 53.36,64.69 53.34,71.29 C1.2 v47.07,65.22 | R2.2 51.09,64.69 53.36,64.69 | 9.93,48.1 JP8.15
  Bottom 0.305: v14.22,65.2 v6.86,65.2 | v9.91,30.65 v12.7,30.65
  Bottom 0.61: v47.07,65.22 v14.22,65.2
RTCK(LPC176?_ONLY)  (via drill 0.6)
  Top 0.305: 18.72,39.27 U$5.100
  Top 0.61: v18.72,43.08 18.72,39.27 | v7.34,43.05 R40.1 JP8.11
  Bottom 0.61: v7.34,43.05 v18.72,43.08
RXD0  (via drill 0.6)  (1 unrouted)
  Top 0.305: U$5.99 19.51,44.27 v16.51,48.94
  Top 0.61: v35.89,53.23 JP9.2 | v83.31,48.69 85.6,47.67 85.6,39.54 IC11.3
  Bottom 0.61: v16.51,48.94 26.42,48.94 30.23,51.99 30.23,53.26 v35.89,53.23 | JP10.8 v83.31,48.69
RXD1  (via drill 0.6)  (1 unrouted)
  Top 0.305: U$5.63 35.1,29.99 36.33,30.76
  Top 0.61: 36.33,30.76 v36.32,32.13 | JP9.5 v43.48,32.13 | v97.64,39.49 IC10.3
  Bottom 0.61: v36.32,32.13 v43.48,32.13 | JP10.5 91.44,47.42 91.44,39.47 v97.64,39.49
RXD2  (via drill 0.6)  (1 unrouted)
  Top 0.305: U$5.49 30.5,23.78
  Top 0.406: v83.31,17.5 83.31,22.53 85.34,23.54 85.34,31.64 IC12.3
  Top 0.61: 30.5,23.78 v30.5,23.87 | JP11.2 v36.99,23.87
  Bottom 0.61: v36.99,23.87 v30.5,23.87 | v83.31,17.5 JP12.8
RXD3  (via drill 0.6)  (1 unrouted)
  Top 0.305: U$5.47 29.5,20.97 30.48,19.99
  Top 0.406: IC13.3 95.5,31.67 95.5,23.54 v90.93,19.99
  Top 0.61: v32.51,19.99 30.48,19.99
  Bottom 0.61: JP11.5 43.51,22.27 32.51,22.27 v32.51,19.99 | v90.93,19.99 JP12.5
SCK  (1 unrouted)
TCK/SWDCLK  (via drill 0.6)  (1 unrouted)
  Top 0.305: v13.95,41.42 13.97,32.94 15.98,34.01 U$5.5
  Top 0.61: R39.2 JP8.9
  Bottom 0.61: v5.33,41.42 v13.95,41.42
TD+  (2 unrouted)
TD-  (2 unrouted)
TDI  (via drill 0.6)
  Top 0.305: U$5.2 16,35.48 v15.24,35.99
  Top 0.61: JP8.5 R37.2 v5.33,34.97
  Bottom 0.61: v5.33,34.97 v15.24,35.99
TDO/SWO  (via drill 0.6)
  Top 0.305: U$5.1 16.51,36.02 v16.51,46.33
  Top 0.61: v5.38,46.35 R41.1 JP8.13
  Bottom 0.61: v5.38,46.35 v16.51,46.33
TMS/SWDIO  (via drill 0.6)  (1 unrouted)
  Top 0.305: U$5.3 18.8,34.97 18.8,36.24 17.78,37.26 v17.75,38.5
  Top 0.61: R38.2 JP8.7
  Bottom 0.61: v7.32,38.5 v17.75,38.5
TRST_N  (via drill 0.6)
  Top 0.305: U$5.4 16.13,34.52 v15.24,34.72
  Top 0.61: v7.29,32.66 R36.2 JP8.3
  Bottom 0.61: v7.29,32.66 v15.24,34.72
TXD0  (via drill 0.6)  (1 unrouted)
  Top 0.305: v18.54,47.67 19.99,44.9 U$5.98
  Top 0.61: v84.58,51.23 87.88,51.23 87.86,43.28 IC11.6
  Bottom 0.61: JP9.1 29.64,49.98 26.59,47.67 v18.54,47.67 | JP10.9 v84.58,51.23
TXD1  (via drill 0.6)  (1 unrouted)
  Top 0.61: JP9.4 40.95,45.79 v40.93,29.5 | v88.9,48.69 97.54,48.69 97.56,43.3 IC10.6
  Bottom 0.61: v36.12,29.49 v40.93,29.5 | JP10.6 v88.9,48.69
TXD2  (via drill 0.6)  (1 unrouted)
  Top 0.305: U$5.48 30,21.23 30.23,21 30.48,21
  Top 0.406: v83.01,23.97 84.33,24.05 84.33,27.86 IC12.6
  Top 0.61: 30.48,21 34.39,21.03 JP11.1
  Bottom 0.61: v83.01,23.97 80.75,23.95 JP12.9
TXD3  (via drill 0.6)  (1 unrouted)
  Top 0.305: U$5.46 29,23.5
  Top 0.406: v88.39,19.22 88.39,21.26 94.74,24.3 94.74,27.86 IC13.6
  Top 0.61: 29,23.5 v28.98,27.38 | v41.99,27.38 JP11.4
  Bottom 0.61: v28.98,27.38 v41.99,27.38 | v88.39,19.22 JP12.6
USB  (2 unrouted)
USB-MODE
  Top 0.61: JP5.1 44.8,63.93 JP4.1
USB_D+  (3 unrouted)
USB_D-  (3 unrouted)
USB_OVRCR  (1 unrouted)
USB_PWRD  (5 unrouted)
USB_UP_LED  (via drill 0.6)  (1 unrouted)
  Top 0.305: U$5.32 22,26.08 v22.1,26.34 | v7.87,26.34 11.68,28.62 11.94,54.28
  Top 0.61: 11.94,54.28 10.67,54.28 v10.67,63.93
  Bottom 0.305: v22.1,26.34 v7.87,26.34
  Bottom 0.61: v10.67,63.93 18.8,63.93 19.3,64.44 22.35,64.44 22.86,63.93 v32.77,63.93
VBUS  (via drill 0.6)  (1 unrouted)
  Top 0.305: U$5.21 14.25,26.01 v14.22,25.32 | v6.86,25.32 10.92,28.37
  Bottom 0.305: v14.22,25.32 v6.86,25.32
VCC  (4 unrouted)
  Top 0.61: IC8.3 20.21,8.86 | 13.59,6.91 13.59,6.59 | 20.73,6.59 20.22,6.59 | 29.72,1.29 IC6.3 | R26.1 15.24,4.99 15.24,6.59 | C20.2 17.27,5.13 17.27,6.59 | C22.2 27.18,2.82
  Top 1.27: X3.1 10.41,16.18 11.68,12.87 13.59,6.91 | 13.59,6.59 15.24,6.59 17.27,6.59 20.22,6.59 20.22,1.29 27.18,1.29 | 20.73,6.59 IC8.3 | 27.18,1.29 29.72,1.29 | 27.18,2.82 27.18,1.29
